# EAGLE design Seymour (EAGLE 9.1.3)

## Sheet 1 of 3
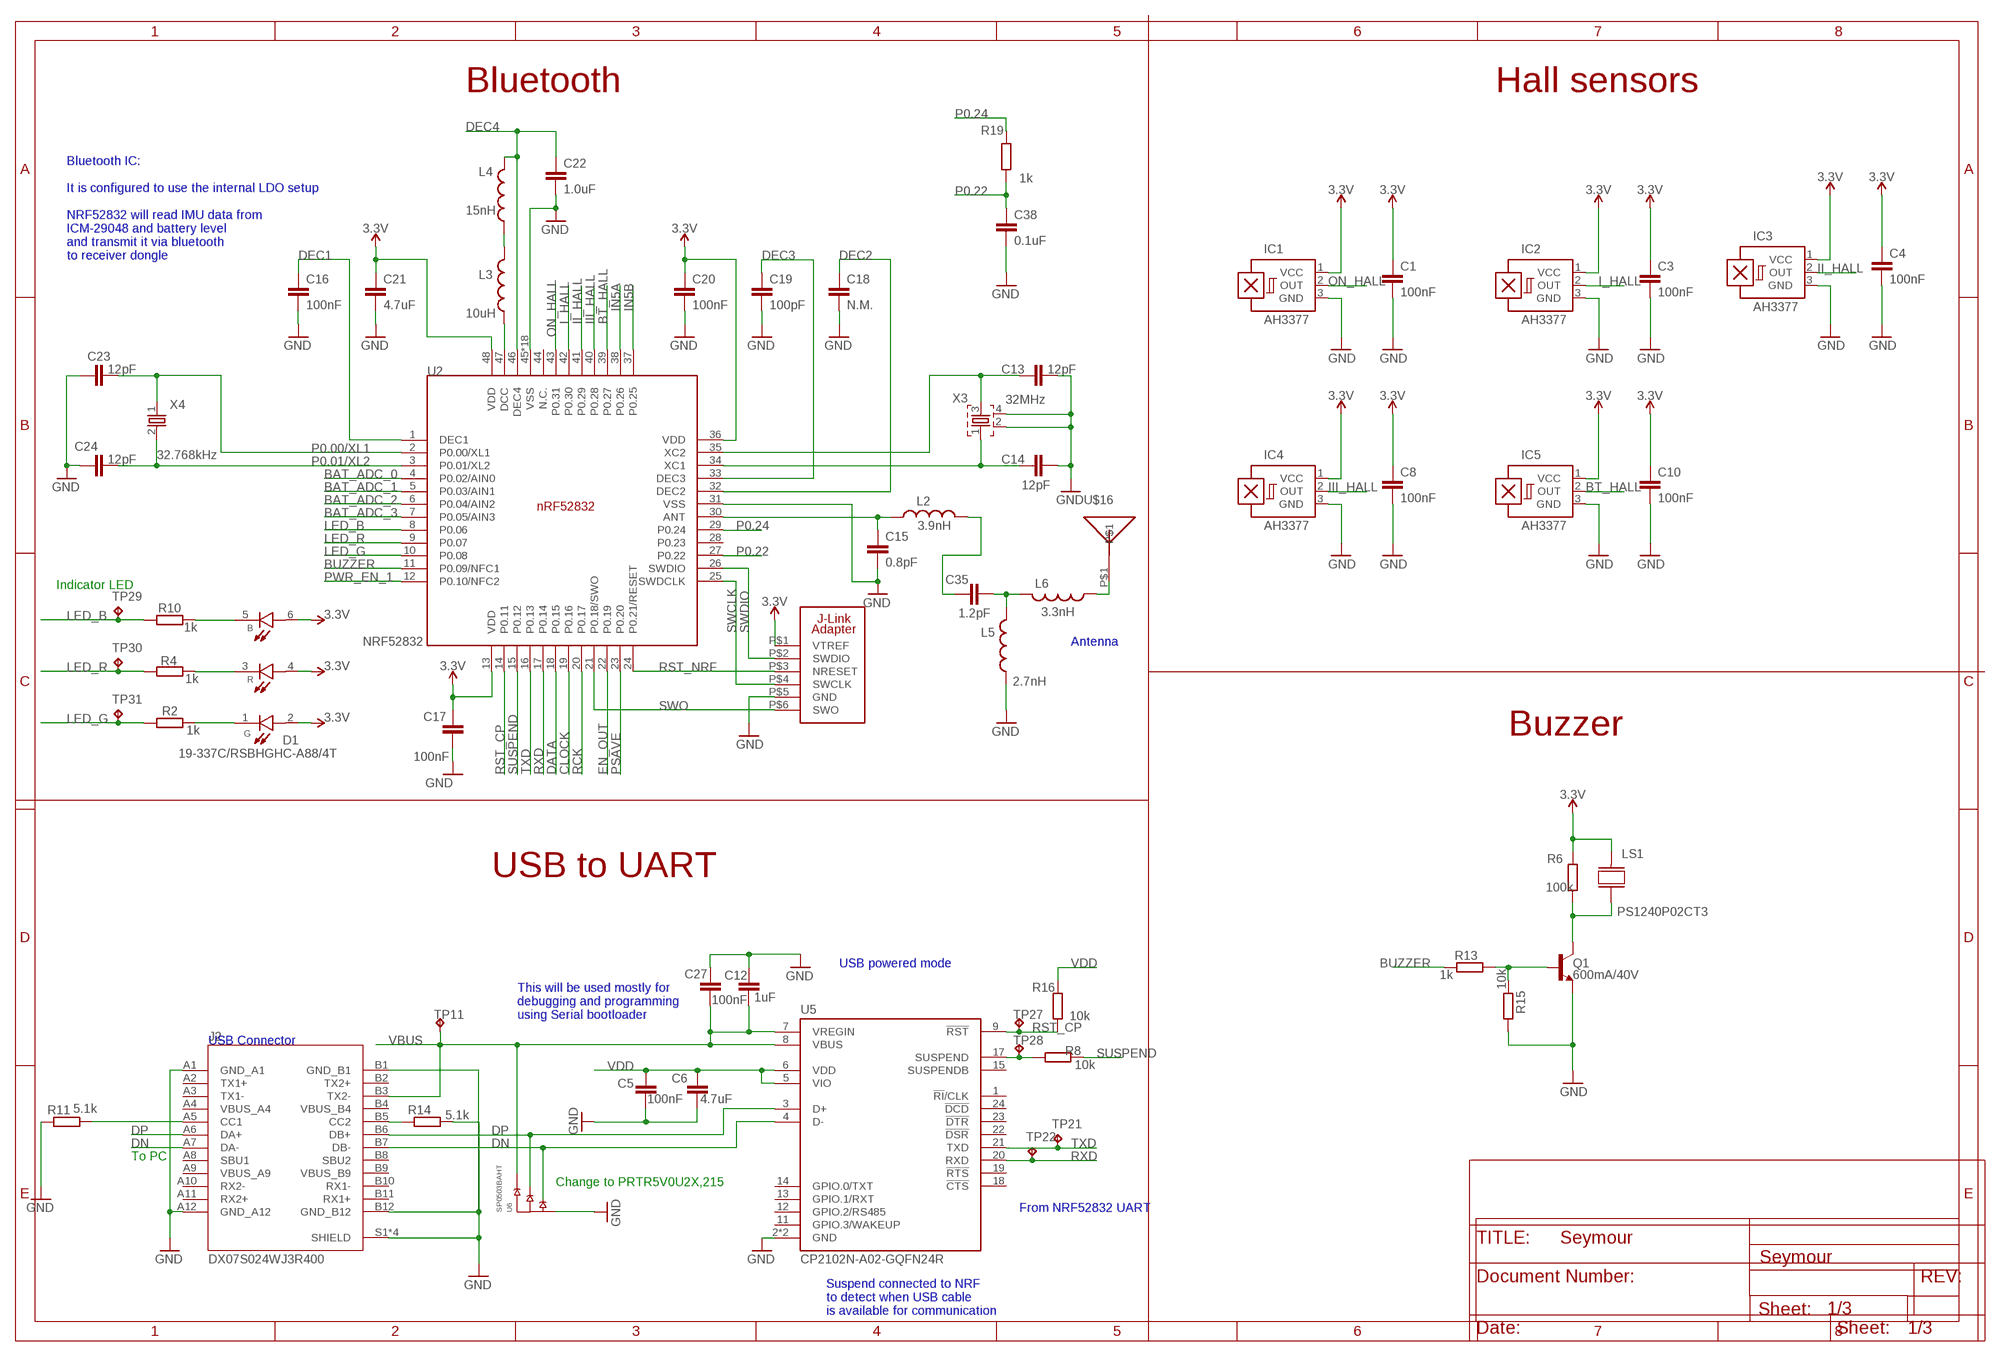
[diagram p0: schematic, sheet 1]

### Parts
C1  100nF  C-EUC0402  [C0402]
C3  100nF  C-EUC0402  [C0402]
C4  100nF  C-EUC0402  [C0402]
C5  100nF  C-EUC0402  [C0402]
C6  4.7uF  C-EUC0603  [C0603]
C8  100nF  C-EUC0402  [C0402]
C10  100nF  C-EUC0402  [C0402]
C12  1uF  C-EUC0603  [C0603]
C13  12pF  C-EUC0402  [C0402]
C14  12pF  C-EUC0402  [C0402]
C15  0.8pF  C-EUC0402  [C0402]
C16  100nF  C-EUC0603  [C0603]
C17  100nF  C-EUC0402  [C0402]
C18  N.M.  C-EUC0603  [C0603]
C19  100pF  C-EUC0402  [C0402]
C20  100nF  C-EUC0402  [C0402]
C21  4.7uF  C-EUC0603  [C0603]
C22  1.0uF  C-EUC0603  [C0603]
C23  12pF  C-EUC0402  [C0402]
C24  12pF  C-EUC0402  [C0402]
C27  100nF  C-EUC0402  [C0402]
C35  1.2pF  CAPACITOR_0402_N  [RESC0402_N]
C38  0.1uF  C-EUC0402  [C0402]
D1  19-337C/RSBHGHC-A88/4T  [LED_19-337C/RSBHGHC-A88/4T]
IC1  AH3377  A1203LH  [SOT23-W]
IC2  AH3377  A1203LH  [SOT23-W]
IC3  AH3377  A1203LH  [SOT23-W]
IC4  AH3377  A1203LH  [SOT23-W]
IC5  AH3377  A1203LH  [SOT23-W]
J2  DX07S024WJ3R400  [JAE_DX07S024WJ3R400]
L2  3.9nH  INDUCTOR_0402_N  [RESC0402_N]
L3  10uH  INDUCTOR_0603_N  [RESC0603_N]
L4  15nH  INDUCTOR_0402_N  [RESC0402_N]
L5  2.7nH  INDUCTOR_0402_N  [RESC0402_N]
L6  3.3nH  INDUCTOR_0402_N  [RESC0402_N]
LS1  PS1240P02CT3  [XDCR_PS1240P02CT3]
Q1  600mA/40V  TRANS_NPN-MMBT2222AL  [SOT23-3]
R2  1k  R-EU_R0402  [R0402]
R4  1k  R-EU_R0402  [R0402]
R6  100k  R-EU_R0402  [R0402]
R8  10k  R-EU_R0402  [R0402]
R10  1k  R-EU_R0402  [R0402]
R11  5.1k  R-EU_R0402  [R0402]
R13  1k  R-EU_R0402  [R0402]
R14  5.1k  R-EU_R0402  [R0402]
R15  10k  R-EU_R0402  [R0402]
R16  10k  R-EU_R0402  [R0402]
R19  1k  R-EU_R0402  [R0402]
TP11  TPTP06R  [TP06R]
TP21  TPTP06R  [TP06R]
TP22  TPTP06R  [TP06R]
TP27  TPTP06R  [TP06R]
TP28  TPTP06R  [TP06R]
TP29  TPTP06R  [TP06R]
TP30  TPTP06R  [TP06R]
TP31  TPTP06R  [TP06R]
U2  NRF52832  [QFN40P600X600X90-48_N]
U5  CP2102N-A02-GQFN24R  [QFN50P400X400X80-25N]
U6  SP0503BAHT  [SOT143]
U$1  J-LINK_6-PIN_ADAPTER-1  [J-LINK_6-PIN_ADAPTER_S]
U$16  ANT_2450AT18B100E  [2450AT18B100E]
X3  32MHz  XTAL_32MHZ  [BT-XTAL_2016_N]
X4  32.768kHz  XTAL_32KHZ  [XTAL_3215_N]

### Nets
3.3V: C1.1 C3.1 C4.1 C8.1 C10.1 C17.1 C20.1 C21.1 D1.2(G_A) D1.4(R_A) D1.6(B_A) IC1.1(VCC) IC2.1(VCC) IC3.1(VCC) IC4.1(VCC) IC5.1(VCC) LS1.2 R6.1 U2.13(VDD) U2.36(VDD) U2.48(VDD) U$1.P$1(VTREF) ; also sheet 2
ANT1: C15.1 L2.1 U2.30(ANT)
BAT_ADC_0: U2.4(P0.02/AIN0) ; also sheet 3
BAT_ADC_1: U2.5(P0.03/AIN1) ; also sheet 3
BAT_ADC_2: U2.6(P0.04/AIN2) ; also sheet 3
BAT_ADC_3: U2.7(P0.05/AIN3) ; also sheet 3
BT_HALL: IC5.2(OUT) U2.39(P0.27)
BUZZER: R13.1 U2.11(P0.09/NFC1)
CLOCK: U2.19(P0.16) ; also sheet 2
DATA: U2.18(P0.15) ; also sheet 2
DEC1: C16.1 U2.1(DEC1)
DEC2: C18.1 U2.32(DEC2)
DEC3: C19.1 U2.33(DEC3)
DEC4: C22.1 L4.2 U2.46(DEC4)
DN: J2.A7(DA-) J2.B7(DB-) U5.4(D-) U6.2(A)
DP: J2.A6(DA+) J2.B6(DB+) U5.3(D+) U6.3(B)
EN_OUT: U2.22(P0.19) ; also sheet 2
GND: C1.2 C3.2 C4.2 C5.1 C6.2 C8.2 C10.2 C12.1 C13.2 C14.2 C15.2 C16.2 C17.2 C18.2 C19.2 C20.2 C21.2 C22.2 C23.1 C24.1 C27.2 C38.2 IC1.3(GND) IC2.3(GND) IC3.3(GND) IC4.3(GND) IC5.3(GND) J2.A1(GND_A1) J2.A12(GND_A12) J2.B1(GND_B1) J2.B12(GND_B12) J2.S1(SHIELD) J2.S2(SHIELD) J2.S3(SHIELD) J2.S4(SHIELD) L5.1 Q1.2(E) R11.1 R14.2 R15.2 U2.31(VSS) U2.45(VSS) U2.PAD(VSS) U2.PAD@VIA01(VSS) U2.PAD@VIA02(VSS) U2.PAD@VIA03(VSS) U2.PAD@VIA04(VSS) U2.PAD@VIA05(VSS) U2.PAD@VIA06(VSS) U2.PAD@VIA07(VSS) U2.PAD@VIA08(VSS) U2.PAD@VIA09(VSS) U2.PAD@VIA10(VSS) U2.PAD@VIA11(VSS) U2.PAD@VIA12(VSS) U2.PAD@VIA13(VSS) U2.PAD@VIA14(VSS) U2.PAD@VIA15(VSS) U2.PAD@VIA16(VSS) U5.2(GND) U5.25(GND) U6.1(GND) U$1.P$5(GND) X3.2 X3.4 ; also sheet 2,3
I_HALL: IC2.2(OUT) U2.42(P0.30)
II_HALL: IC3.2(OUT) U2.41(P0.29)
III_HALL: IC4.2(OUT) U2.40(P0.28)
IN5A: U2.38(P0.26) ; also sheet 2
IN5B: U2.37(P0.25) ; also sheet 2
LED_B: R10.2 TP29.TP U2.8(P0.06)
LED_G: R2.2 TP31.TP U2.10(P0.08)
LED_R: R4.2 TP30.TP U2.9(P0.07) ; also sheet 3
N$1: C13.1 U2.35(XC2) X3.3
N$2: C35.2 L2.2
N$3: R8.1 TP28.TP U5.17(SUSPEND)
N$4: J2.A5(CC1) R11.2
N$5: J2.B5(CC2) R14.1
N$8: D1.3(R_C) R4.1
N$10: D1.5(B_C) R10.1
N$14: Q1.1(B) R13.2 R15.1
N$15: D1.1(G_C) R2.1
N$16: LS1.1 Q1.3(C) R6.2
N$17: L3.1 U2.47(DCC)
N$20: L3.2 L4.1
N$29: C35.1 L5.2 L6.2
N$30: L6.1 U$16.P$1
ON_HALL: IC1.2(OUT) U2.43(P0.31)
P0.00/XL1: C23.2 U2.2(P0.00/XL1) X4.1
P0.01/XL2: C24.2 U2.3(P0.01/XL2) X4.2
P0.22: C38.1 R19.1 U2.27(P0.22)
P0.24: R19.2 U2.29(P0.24)
PSAVE: U2.23(P0.20) ; also sheet 2
PWR_EN_1: U2.12(P0.10/NFC2) ; also sheet 2
RCK: U2.20(P0.17) ; also sheet 2
RST_CP: R16.2 TP27.TP U2.14(P0.11) U5.9(!RST)
RST_NRF: U2.24(P0.21/RESET) U$1.P$3(NRESET)
RXD: TP22.TP U2.17(P0.14) U5.20(RXD)
SUSPEND: R8.2 U2.15(P0.12)
SWCLK: U2.25(SWDCLK) U$1.P$4(SWCLK)
SWDIO: U2.26(SWDIO) U$1.P$2(SWDIO)
SWO: U2.21(P0.18/SWO) U$1.P$6(SWO)
TXD: TP21.TP U2.16(P0.13) U5.21(TXD)
VBUS: C12.2 C27.1 J2.B3(TX2-) TP11.TP U5.7(VREGIN) U5.8(VBUS) U6.4(C) ; also sheet 3
VDD: C5.2 C6.1 R16.1 U5.5(VIO) U5.6(VDD)
X2: C14.1 U2.34(XC1) X3.1
Unconnected: J2.A2(TX1+) J2.A3(TX1-) J2.A4(VBUS_A4) J2.A8(SBU1) J2.A9(VBUS_A9) J2.A10(RX2-) J2.A11(RX2+) J2.B2(TX2+) J2.B4(VBUS_B4) J2.B8(SBU2) J2.B9(VBUS_B9) J2.B10(RX1-) J2.B11(RX1+) U2.28(P0.23) U2.44(N.C.) U5.1(!RI!/CLK) U5.11(GPIO.3/WAKEUP) U5.12(GPIO.2/RS485) U5.13(GPIO.1/RXT) U5.14(GPIO.0/TXT) U5.15(SUSPENDB) U5.18(!CTS) U5.19(!RTS) U5.22(!DSR) U5.23(!DTR) U5.24(!DCD)

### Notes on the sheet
- Bluetooth | Hall sensors
- 1k
- Bluetooth IC:
  
  It is configured to use the internal LDO setup
  
  NRF52832 will read IMU data from 
  ICM-29048 and battery level 
  and transmit it via bluetooth 
  to receiver dongle
- Indicator LED
- Antenna
- Buzzer
- USB to UART
- USB powered mode
- This will be used mostly for 
  debugging and programming 
  using Serial bootloader
- USB Connector
- To PC
- Change to PRTR5V0U2X,215‎
- From NRF52832 UART
- Suspend connected to NRF 
  to detect when USB cable 
  is available for communication

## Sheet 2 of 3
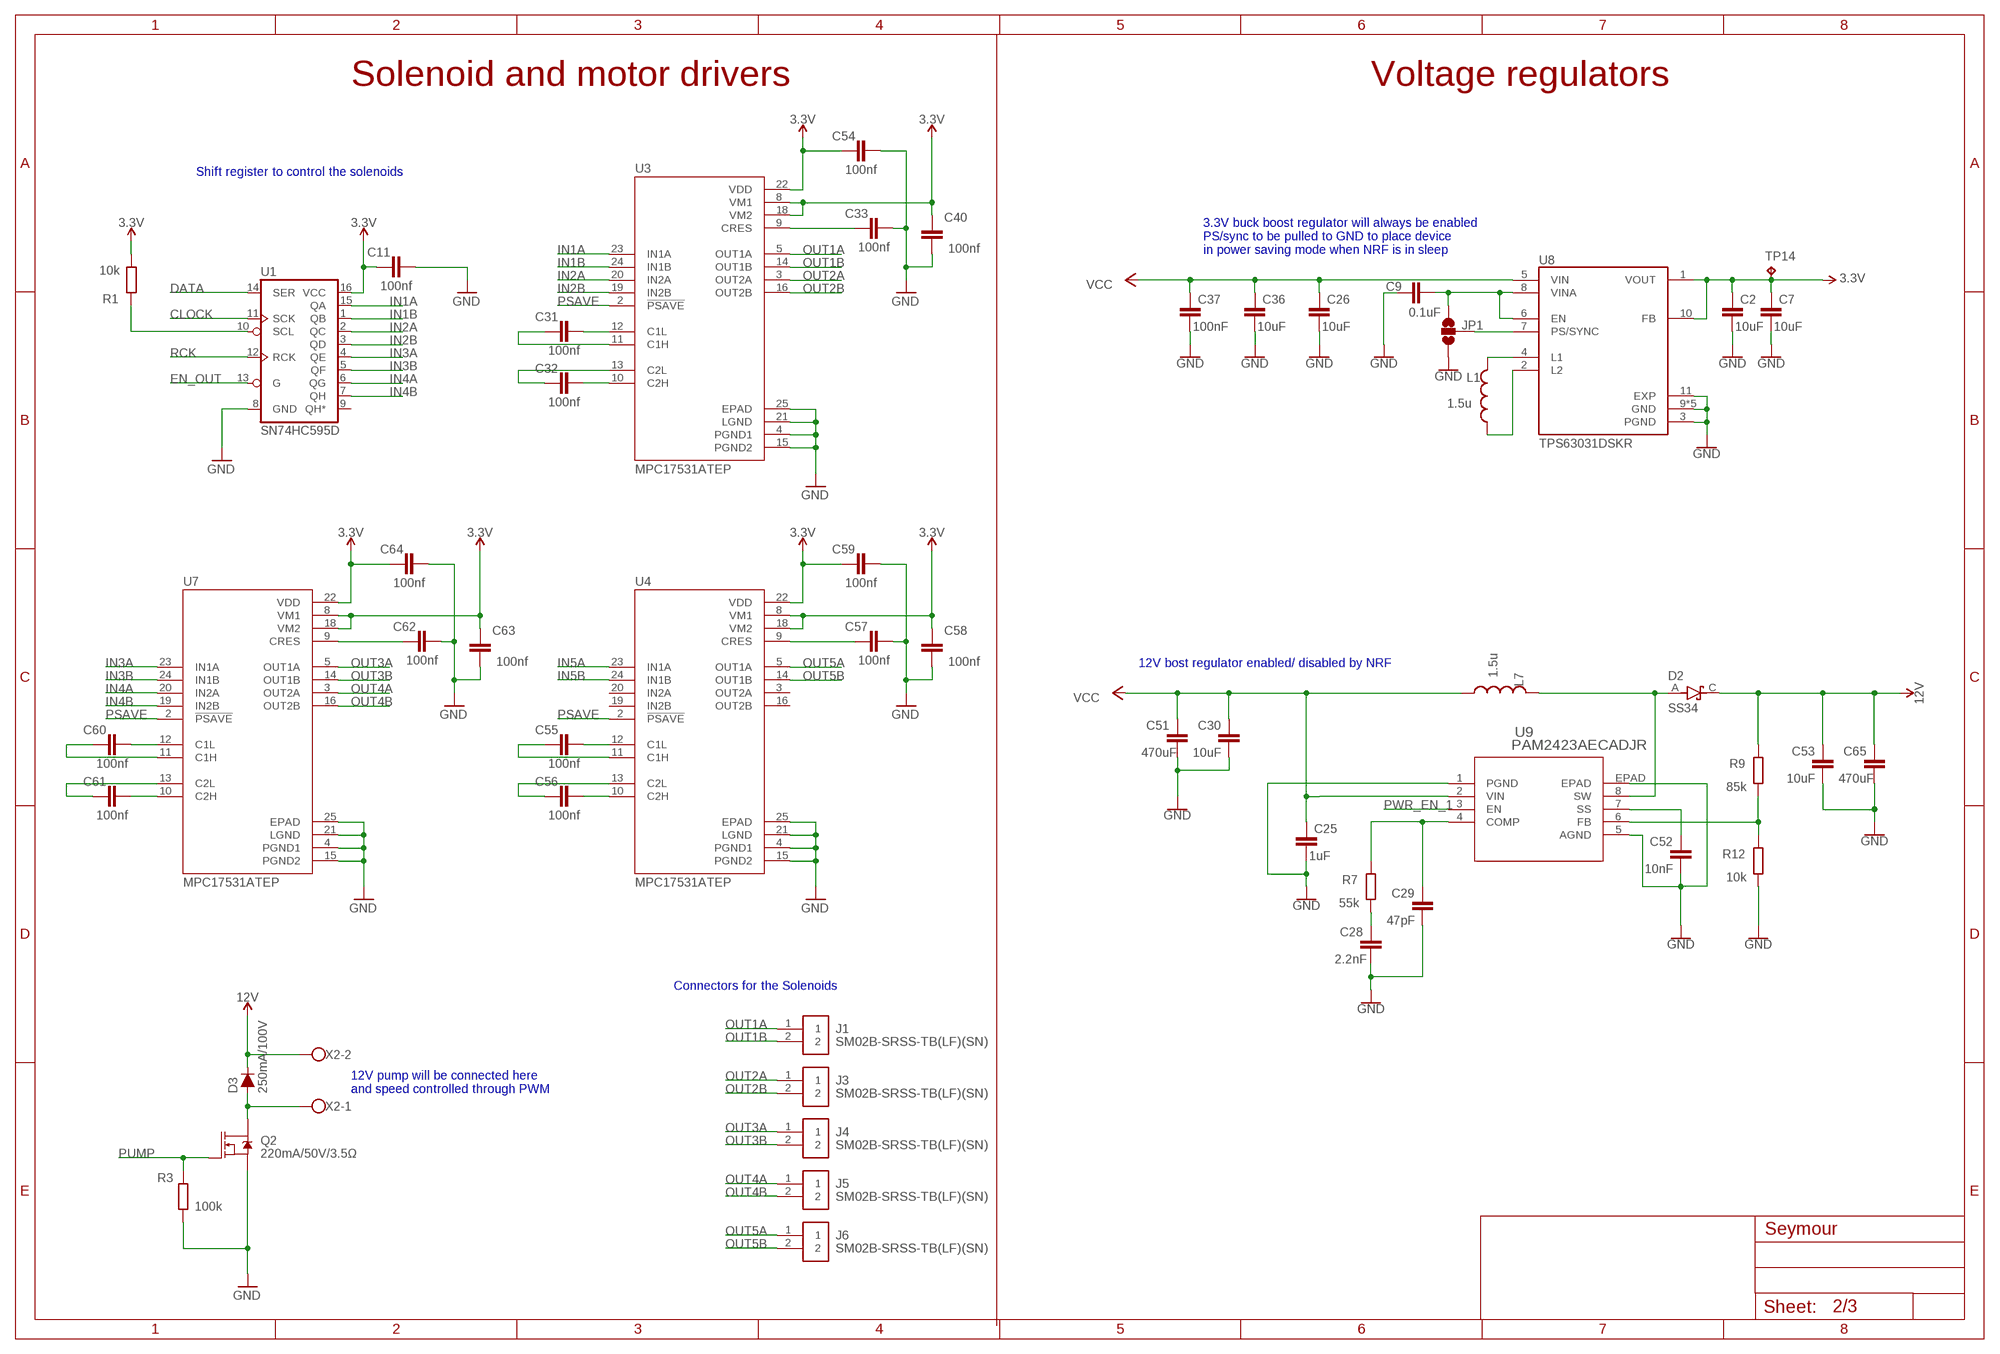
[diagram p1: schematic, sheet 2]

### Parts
C2  10uF  C-EUC0603  [C0603]
C7  10uF  C-EUC0603  [C0603]
C9  0.1uF  C-EUC0603  [C0603]
C11  100nf  CAPACITOR_0402_N  [RESC0402_N]
C25  1uF  C-EUC0603  [C0603]
C26  10uF  C-EUC0603  [C0603]
C28  2.2nF  C-EUC0603  [C0603]
C29  47pF  C-EUC0603  [C0603]
C30  10uF  C-EUC0603  [C0603]
C31  100nf  CAPACITOR_0402_N  [RESC0402_N]
C32  100nf  CAPACITOR_0402_N  [RESC0402_N]
C33  100nf  CAPACITOR_0402_N  [RESC0402_N]
C36  10uF  C-EUC0603  [C0603]
C37  100nF  C-EUC0603  [C0603]
C40  100nf  CAPACITOR_0402_N  [RESC0402_N]
C51  470uF  C-EUC0603  [C0603]
C52  10nF  C-EUC0603  [C0603]
C53  10uF  C-EUC0603  [C0603]
C54  100nf  CAPACITOR_0402_N  [RESC0402_N]
C55  100nf  CAPACITOR_0402_N  [RESC0402_N]
C56  100nf  CAPACITOR_0402_N  [RESC0402_N]
C57  100nf  CAPACITOR_0402_N  [RESC0402_N]
C58  100nf  CAPACITOR_0402_N  [RESC0402_N]
C59  100nf  CAPACITOR_0402_N  [RESC0402_N]
C60  100nf  CAPACITOR_0402_N  [RESC0402_N]
C61  100nf  CAPACITOR_0402_N  [RESC0402_N]
C62  100nf  CAPACITOR_0402_N  [RESC0402_N]
C63  100nf  CAPACITOR_0402_N  [RESC0402_N]
C64  100nf  CAPACITOR_0402_N  [RESC0402_N]
C65  470uF  C-EUC0603  [C0603]
D2  SS34  [DIOM7959X265N]
D3  250mA/100V  DIODE-BAS16J  [SOD-323]
J1  SM02B-SRSS-TB(LF)(SN)  [SM02B-SRSS-TB(LF)(SN)]
J3  SM02B-SRSS-TB(LF)(SN)  [SM02B-SRSS-TB(LF)(SN)]
J4  SM02B-SRSS-TB(LF)(SN)  [SM02B-SRSS-TB(LF)(SN)]
J5  SM02B-SRSS-TB(LF)(SN)  [SM02B-SRSS-TB(LF)(SN)]
J6  SM02B-SRSS-TB(LF)(SN)  [SM02B-SRSS-TB(LF)(SN)]
JP1  SPARKFUN-JUMPERS_JUMPER-SMT_NC  [SPARKFUN-JUMPERS_SMT-JUMPER_TRACE_SILK]
L1  1.5u  XFL4020  [XFL4020]
L7  1.5u  XFL4020  [XFL4020]
Q2  220mA/50V/3.5Ω  MOSFET-NCH-BSS138  [SOT23-3]
R1  10k  R-EU_R0402  [R0402]
R3  100k  R-EU_R0402  [R0402]
R7  55k  R-EU_R0402  [R0402]
R9  85k  R-EU_R0402  [R0402]
R12  10k  R-EU_R0402  [R0402]
TP14  TPTP06R  [TP06R]
U1  SN74HC595D  74HC595D  [SO16]
U3  MPC17531ATEP  [QFN50P400X400X100-25N]
U4  MPC17531ATEP  [QFN50P400X400X100-25N]
U7  MPC17531ATEP  [QFN50P400X400X100-25N]
U8  TPS63031DSKR  [SON50P250X250X80-11N]
U9  PAM2423AECADJR  [SOP-8_PAM2423AECADJR_DIO]
X2  W237-102  [W237-102]

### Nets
3.3V: C2.1 C7.1 C11.2 C40.1 C54.2 C58.1 C59.2 C63.1 C64.2 R1.2 TP14.TP U1.16(VCC) U3.8(VM1) U3.18(VM2) U3.22(VDD) U4.8(VM1) U4.18(VM2) U4.22(VDD) U7.8(VM1) U7.18(VM2) U7.22(VDD) U8.1(VOUT) U8.10(FB) ; also sheet 1
12V: C53.1 C65.1 D2.C(K) D3.C R9.2 X2.2
CLOCK: U1.11(SCK) ; also sheet 1
DATA: U1.14(SER) ; also sheet 1
EN_OUT: U1.13(G) ; also sheet 1
GND: C2.2 C7.2 C9.1 C11.1 C25.2 C26.2 C28.2 C29.2 C30.2 C33.1 C36.2 C37.2 C40.2 C51.2 C52.2 C53.2 C54.1 C57.1 C58.2 C59.1 C62.1 C63.2 C64.1 C65.2 JP1.1 Q2.2(S) R3.2 R12.1 U1.8(GND) U3.4(PGND1) U3.15(PGND2) U3.21(LGND) U3.25(EPAD) U4.4(PGND1) U4.15(PGND2) U4.21(LGND) U4.25(EPAD) U7.4(PGND1) U7.15(PGND2) U7.21(LGND) U7.25(EPAD) U8.3(PGND) U8.9(GND) U8.11(EXP) U8.12(GND) U8.13(GND) U8.14(GND) U8.15(GND) U9.1(PGND) U9.5(AGND) U9.EPAD ; also sheet 1,3
IN1A: U1.15(QA) U3.23(IN1A)
IN1B: U1.1(QB) U3.24(IN1B)
IN2A: U1.2(QC) U3.20(IN2A)
IN2B: U1.3(QD) U3.19(IN2B)
IN3A: U1.4(QE) U7.23(IN1A)
IN3B: U1.5(QF) U7.24(IN1B)
IN4A: U1.6(QG) U7.20(IN2A)
IN4B: U1.7(QH) U7.19(IN2B)
IN5A: U4.23(IN1A) ; also sheet 1
IN5B: U4.24(IN1B) ; also sheet 1
N$6: C9.2 JP1.3 U8.6(EN) U8.8(VINA)
N$7: L1.P$2 U8.4(L1)
N$9: R1.1 U1.10(SCL)
N$11: L1.P$1 U8.2(L2)
N$12: D2.A L7.P$2 U9.8(SW)
N$13: JP1.2 U8.7(PS/SYNC)
N$18: C29.1 R7.2 U9.4(COMP)
N$19: C28.1 R7.1
N$23: C52.1 U9.7(SS)
N$39: R9.1 R12.2 U9.6(FB)
N$43: C32.1 U3.10(C2H)
N$44: C32.2 U3.13(C2L)
N$45: C31.2 U3.11(C1H)
N$46: C31.1 U3.12(C1L)
N$47: C33.2 U3.9(CRES)
N$48: D3.A Q2.3(D) X2.1
N$51: C56.1 U4.10(C2H)
N$52: C56.2 U4.13(C2L)
N$53: C55.2 U4.11(C1H)
N$54: C55.1 U4.12(C1L)
N$55: C57.2 U4.9(CRES)
N$58: C61.1 U7.10(C2H)
N$59: C61.2 U7.13(C2L)
N$60: C60.2 U7.11(C1H)
N$61: C60.1 U7.12(C1L)
N$62: C62.2 U7.9(CRES)
OUT1A: J1.1 U3.5(OUT1A)
OUT1B: J1.2 U3.14(OUT1B)
OUT2A: J3.1 U3.3(OUT2A)
OUT2B: J3.2 U3.16(OUT2B)
OUT3A: J4.1 U7.5(OUT1A)
OUT3B: J4.2 U7.14(OUT1B)
OUT4A: J5.1 U7.3(OUT2A)
OUT4B: J5.2 U7.16(OUT2B)
OUT5A: J6.1 U4.5(OUT1A)
OUT5B: J6.2 U4.14(OUT1B)
PSAVE: U3.2(!PSAVE) U4.2(!PSAVE) U7.2(!PSAVE) ; also sheet 1
PUMP: Q2.1(G) R3.1
PWR_EN_1: U9.3(EN) ; also sheet 1
RCK: U1.12(RCK) ; also sheet 1
VCC: C25.1 C26.1 C30.1 C36.1 C37.1 C51.1 L7.P$1 U8.5(VIN) U9.2(VIN) ; also sheet 3
Unconnected: U1.9(QH*) U4.3(OUT2A) U4.16(OUT2B) U4.19(IN2B) U4.20(IN2A)

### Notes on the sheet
- Solenoid and motor drivers | Voltage regulators
- Shift register to control the solenoids
- 3.3V buck boost regulator will always be enabled
  PS/sync to be pulled to GND to place device 
  in power saving mode when NRF is in sleep
- 12V bost regulator enabled/ disabled by NRF
- Connectors for the Solenoids
- 12V pump will be connected here 
  and speed controlled through PWM

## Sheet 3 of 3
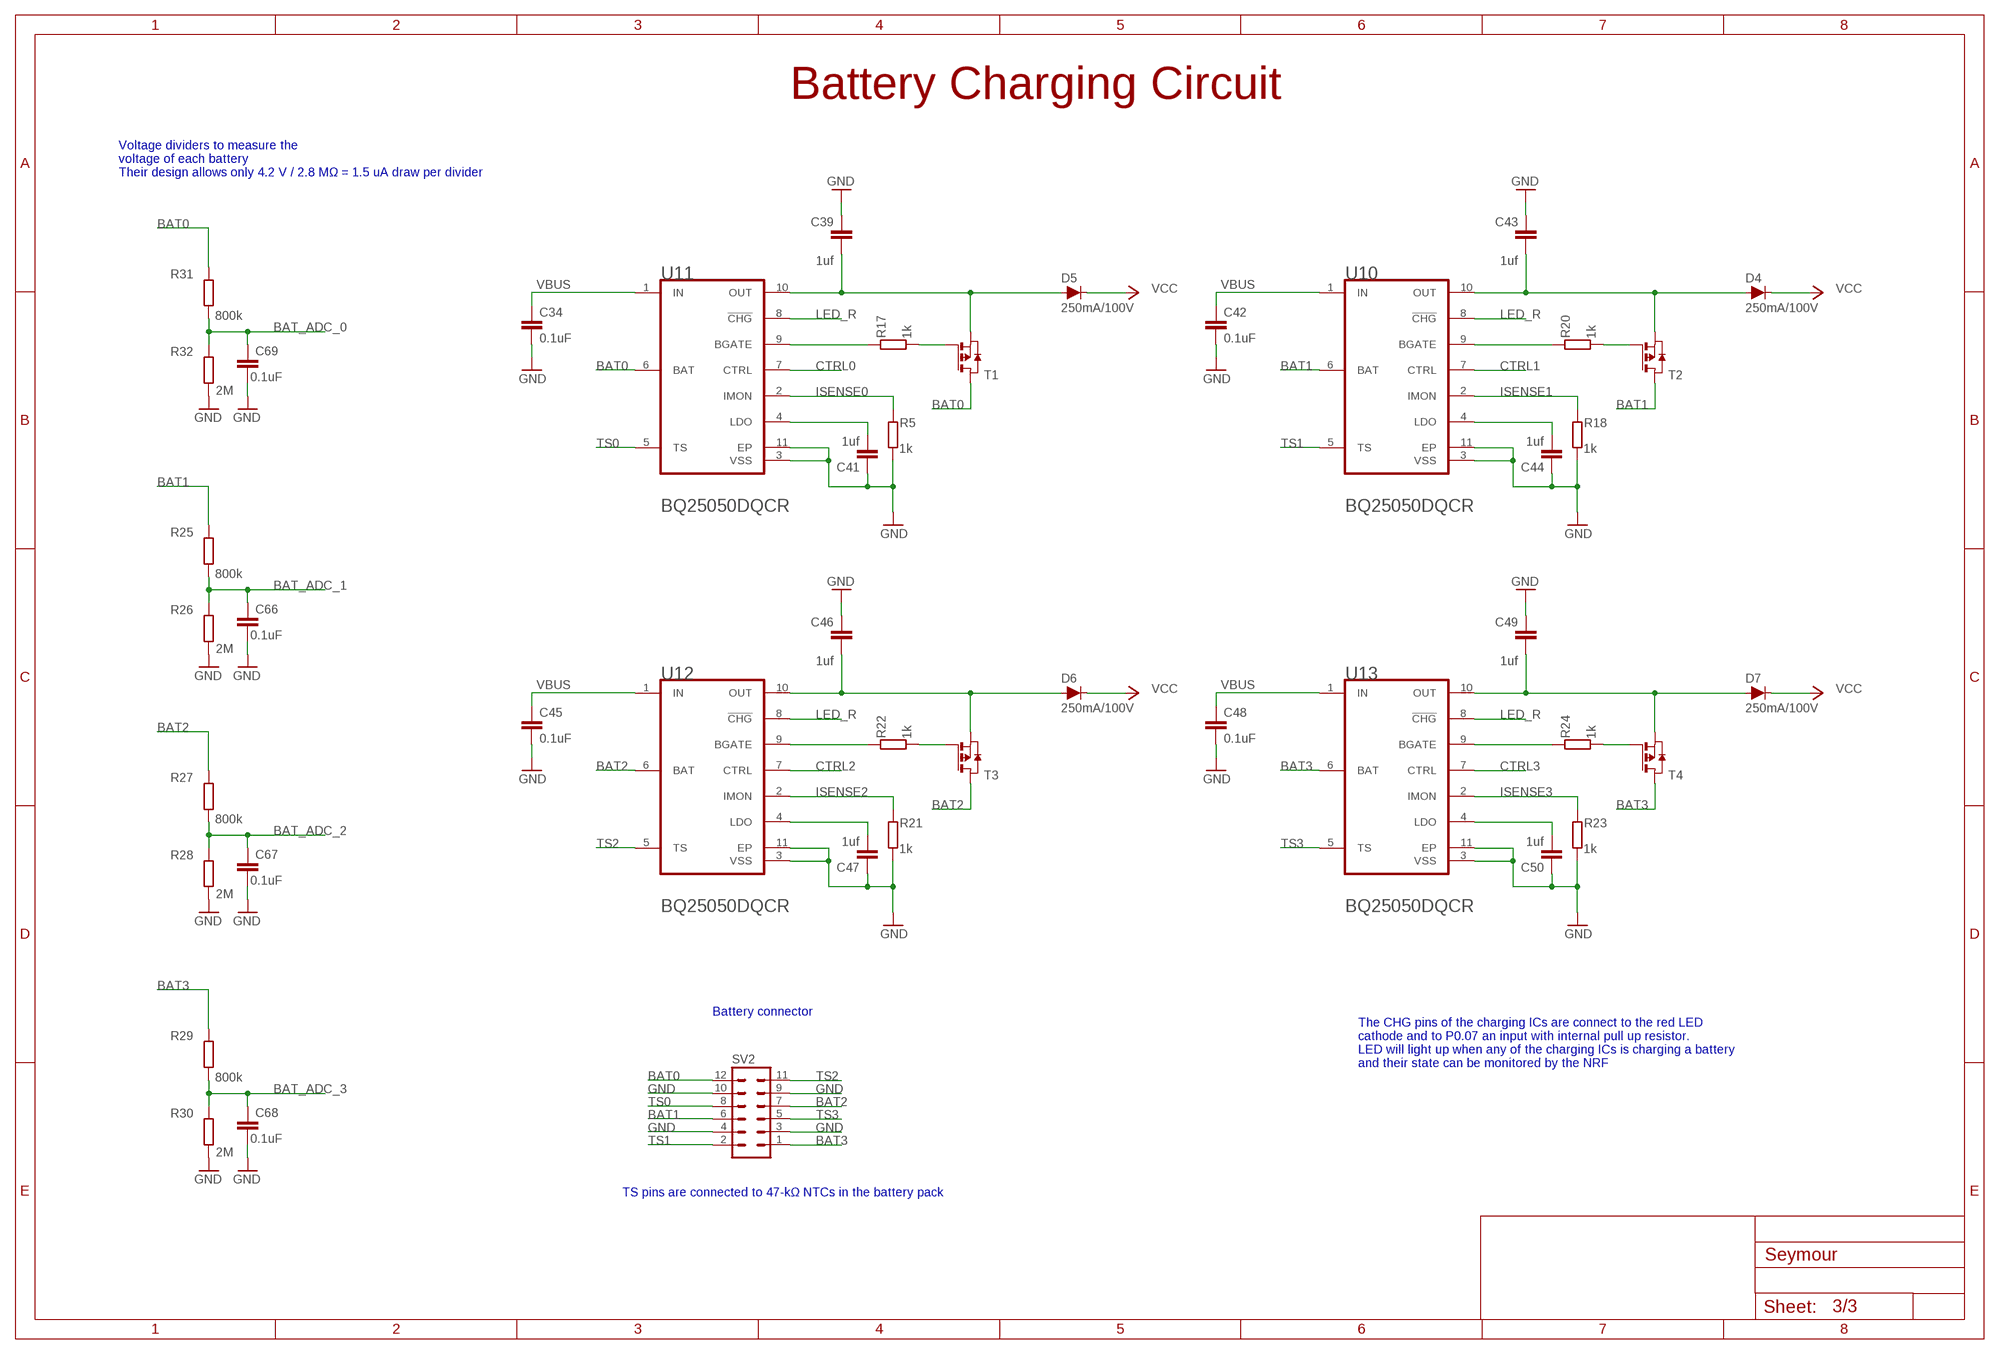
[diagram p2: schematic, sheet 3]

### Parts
C34  0.1uF  C-EUC0402  [C0402]
C39  1uf  C-EUC0402  [C0402]
C41  1uf  C-EUC0402  [C0402]
C42  0.1uF  C-EUC0402  [C0402]
C43  1uf  C-EUC0402  [C0402]
C44  1uf  C-EUC0402  [C0402]
C45  0.1uF  C-EUC0402  [C0402]
C46  1uf  C-EUC0402  [C0402]
C47  1uf  C-EUC0402  [C0402]
C48  0.1uF  C-EUC0402  [C0402]
C49  1uf  C-EUC0402  [C0402]
C50  1uf  C-EUC0402  [C0402]
C66  0.1uF  C-EUC0402  [C0402]
C67  0.1uF  C-EUC0402  [C0402]
C68  0.1uF  C-EUC0402  [C0402]
C69  0.1uF  C-EUC0402  [C0402]
D4  250mA/100V  DIODE-BAS16J  [SOD-323]
D5  250mA/100V  DIODE-BAS16J  [SOD-323]
D6  250mA/100V  DIODE-BAS16J  [SOD-323]
D7  250mA/100V  DIODE-BAS16J  [SOD-323]
R5  1k  R-EU_R0402  [R0402]
R17  1k  R-EU_R0402  [R0402]
R18  1k  R-EU_R0402  [R0402]
R20  1k  R-EU_R0402  [R0402]
R21  1k  R-EU_R0402  [R0402]
R22  1k  R-EU_R0402  [R0402]
R23  1k  R-EU_R0402  [R0402]
R24  1k  R-EU_R0402  [R0402]
R25  800k  R-EU_R0402  [R0402]
R26  2M  R-EU_R0402  [R0402]
R27  800k  R-EU_R0402  [R0402]
R28  2M  R-EU_R0402  [R0402]
R29  800k  R-EU_R0402  [R0402]
R30  2M  R-EU_R0402  [R0402]
R31  800k  R-EU_R0402  [R0402]
R32  2M  R-EU_R0402  [R0402]
SV2  MA06-2  [MA06-2]
T1  PMOSSOT23  [SOT-23]
T2  PMOSSOT23  [SOT-23]
T3  PMOSSOT23  [SOT-23]
T4  PMOSSOT23  [SOT-23]
U10  TEXAS_INSTRUMENTS_BQ25050DQCRTEXAS_INSTRUMENTS_BQ25050DQCR_0_0  [TEXAS_INSTRUMENTS_BQ25050DQCR_0]
U11  TEXAS_INSTRUMENTS_BQ25050DQCRTEXAS_INSTRUMENTS_BQ25050DQCR_0_0  [TEXAS_INSTRUMENTS_BQ25050DQCR_0]
U12  TEXAS_INSTRUMENTS_BQ25050DQCRTEXAS_INSTRUMENTS_BQ25050DQCR_0_0  [TEXAS_INSTRUMENTS_BQ25050DQCR_0]
U13  TEXAS_INSTRUMENTS_BQ25050DQCRTEXAS_INSTRUMENTS_BQ25050DQCR_0_0  [TEXAS_INSTRUMENTS_BQ25050DQCR_0]

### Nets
BAT0: R31.2 SV2.12 T1.1(D) U11.6(BAT)
BAT1: R25.2 SV2.6 T2.1(D) U10.6(BAT)
BAT2: R27.2 SV2.7 T3.1(D) U12.6(BAT)
BAT3: R29.2 SV2.1 T4.1(D) U13.6(BAT)
BAT_ADC_0: C69.1 R31.1 R32.2 ; also sheet 1
BAT_ADC_1: C66.1 R25.1 R26.2 ; also sheet 1
BAT_ADC_2: C67.1 R27.1 R28.2 ; also sheet 1
BAT_ADC_3: C68.1 R29.1 R30.2 ; also sheet 1
CTRL0: U11.7(CTRL)
CTRL1: U10.7(CTRL)
CTRL2: U12.7(CTRL)
CTRL3: U13.7(CTRL)
GND: C34.2 C39.1 C41.1 C42.2 C43.1 C44.1 C45.2 C46.1 C47.1 C48.2 C49.1 C50.1 C66.2 C67.2 C68.2 C69.2 R5.1 R18.1 R21.1 R23.1 R26.1 R28.1 R30.1 R32.1 SV2.3 SV2.4 SV2.9 SV2.10 U10.3(VSS) U10.11(EP) U11.3(VSS) U11.11(EP) U12.3(VSS) U12.11(EP) U13.3(VSS) U13.11(EP) ; also sheet 1,2
ISENSE0: R5.2 U11.2(IMON)
ISENSE1: R18.2 U10.2(IMON)
ISENSE2: R21.2 U12.2(IMON)
ISENSE3: R23.2 U13.2(IMON)
LED_R: U10.8(!CHG!) U11.8(!CHG!) U12.8(!CHG!) U13.8(!CHG!) ; also sheet 1
N$21: R17.1 T1.3(G)
N$24: R17.2 U11.9(BGATE)
N$26: C39.2 D5.A T1.2(S) U11.10(OUT)
N$27: C44.2 U10.4(LDO)
N$28: C41.2 U11.4(LDO)
N$31: C43.2 D4.A T2.2(S) U10.10(OUT)
N$33: R20.2 U10.9(BGATE)
N$34: R20.1 T2.3(G)
N$36: C47.2 U12.4(LDO)
N$37: C46.2 D6.A T3.2(S) U12.10(OUT)
N$40: R22.2 U12.9(BGATE)
N$41: R22.1 T3.3(G)
N$50: C50.2 U13.4(LDO)
N$56: C49.2 D7.A T4.2(S) U13.10(OUT)
N$63: R24.2 U13.9(BGATE)
N$64: R24.1 T4.3(G)
TS0: SV2.8 U11.5(TS)
TS1: SV2.2 U10.5(TS)
TS2: SV2.11 U12.5(TS)
TS3: SV2.5 U13.5(TS)
VBUS: C34.1 C42.1 C45.1 C48.1 U10.1(IN) U11.1(IN) U12.1(IN) U13.1(IN) ; also sheet 1
VCC: D4.C D5.C D6.C D7.C ; also sheet 2

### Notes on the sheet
- Battery Charging Circuit
- Voltage dividers to measure the
  voltage of each battery
  Their design allows only 4.2 V / 2.8 MΩ = 1.5 uA draw per divider
- Battery connector
- The CHG pins of the charging ICs are connect to the red LED
  cathode and to P0.07 an input with internal pull up resistor.
  LED will light up when any of the charging ICs is charging a battery
  and their state can be monitored by the NRF
- TS pins are connected to 47-kΩ NTCs in the battery pack

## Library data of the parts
C1 C3 C4 C8 C10 C17 C20 C34 C39 C41-C50 C66-C69 = rcl:C-EU: CAPACITOR, European symbol; SPICEPREFIX: C
C2 C5-C7 C9 C12-C16 C18 C19 C21-C30 C36-C38 C51-C53 C65 = resistor:C-EU: CAPACITOR, European symbol
C11 C31-C33 C35 C40 C54-C64 = Nordic_nRF:CAPACITOR: Generic chip capacitor
D1 = led:19-337C/RSBHGHC-A88/4T: Red, Green, Blue (RGB) 625nm Red, 530nm Green, 470nm Blue LED Indication - Discrete 2.05V Red, 2.9V Green, 2.9V Blue 0606 (1616 Metric) Check prices; AVAILABILITY: Warning; DESCRIPTION: Red, Green, Blue (RGB) 625nm Red, 530nm Green, 470nm Blue LED Indication - Discrete 2.05V Red, 2.9V Green, 2.9V Blue 0606 (1616 Metric); MF: Everlight Electronics Co Ltd; MP: 19-337C/RSBHGHC-A88/4T; PACKAGE: 0606 Everlight Electronics Co Ltd; PRICE: None; PURCHASE-URL: https://pricing.snapeda.com/search/part/19-337C/RSBHGHC-A88/4T/?ref=eda
D2 = SS34:SS34: Diode Schottky 40V 3A 2-Pin SMC T/R Check prices; AVAILABILITY: In Stock; DESCRIPTION: Diode Schottky 40V 3A Surface Mount SMC (DO-214AB); MF: ON Semiconductor; MP: SS34; PACKAGE: SMC-2 ON Semiconductor; PRICE: None; PURCHASE-URL: https://pricing.snapeda.com/search/part/SS34/?ref=eda
D3-D7 = SparkFun-DiscreteSemi:DIODE: Diode; PROD_ID: DIO-09646
IC1-IC5 = allegro:A12*?: Hall-effect bipolar switch Source: http://www.allegromicro.com/en/Products/Part_Numbers/1202/1202.pdf; MF: ALLEGRO MICROSYSTEMS, INC.; MPN: A1203LLHLT-T; OC_FARNELL: 1791384; OC_NEWARK: 31K6608
J1 J3-J6 = SM02B-SRSS-TB_LF__SN_:SM02B-SRSS-TB(LF)(SN): JST (JAPAN SOLDERLESS TERMINALS) - SM02B-SRSS-TB (LF)(SN) - HEADER, R/A, 2WAY; AVAILABILITY: Unavailable; DESCRIPTION: Connector Header Surface Mount, Right Angle 2 position 0.039 _1.00mm_; MF: JST Sales; MP: SM02B-SRSS-TB_LF__SN_; PACKAGE: None; PRICE: None
J2 = DX07S024WJ3R400:DX07S024WJ3R400: Conn Rcpt Usb3.1 Typec Smd Vert; DESCRIPTION: USB-C (USB TYPE-C) USB 3.2 Gen 2 (USB 3.1 Gen 2, Superspeed + (USB 3.1)) Receptacle Connector 24 Position Surface Mount, Through Hole; DIGI-KEY_PART_NUMBER: 670-2950-1-ND; MF: JAE Electronics; MP: DX07S024WJ3R400; PACKAGE: None; PURCHASE-URL: https://pricing.snapeda.com/search/part/DX07S024WJ3R400/?ref=eda
JP1 = DECAMove:SPARKFUN-JUMPERS_JUMPER-SMT: Normally closed trace jumper (1 of 2 connections) This jumper has a trace between two pads so it's normally closed (NC). The other connection is normally open (NO). Use a razor knife to open the connection. For best results follow the IPC guidelines for cutting traces: Cutout at least 0.063 mm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
L1 L7 = inductor-coilcraft:XFL4020: Coilcraft shielded 4x4mm high temperature inductor
L2-L6 = Nordic_nRF:INDUCTOR: Generic chip inductor
LS1 = PS1240P02CT3:PS1240P02CT3: Buzzers Transducer, Externally Driven Piezo 3V 4kHz 60dB @ 3V, 10cm Through Hole PC Pins; DESCRIPTION: Buzzers Transducer, Externally Driven Piezo 3V 4kHz 60dB @ 3V, 10cm Through Hole PC Pins; DIGI-KEY_PART_NUMBER: 445-5229-1-ND; MF: TDK; MP: PS1240P02CT3; PACKAGE: SIP-5 TDK; PURCHASE-URL: https://pricing.snapeda.com/search/part/PS1240P02CT3/?ref=eda
Q1 = SparkFun-DiscreteSemi:TRANS_NPN: NPN transistor Current controlled devices typically used to amplify current or used as a switch. BC547 - COM-08928 (TO-92 45V 100mA) (1.Collector 2.Base 3.Emitter) 2N3904 - COM-00521 (TO-92 40V 200mA) (1.Emitter 2.Base 3.Collector) P2N2222A - COM-12852 (TO-92 40V 600mA) (1.Collector 2.Base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; PROD_ID: TRANS-08049
Q2 = SparkFun-DiscreteSemi:MOSFET-NCH: N-channel MOSFETs Voltage controlled devices that allow control of high current outputs. SparkFun Products: SparkFun OpenScale SparkFun Digital Sandbox SparkFun Monster Moto Shield SparkFun MOSFET Power Controller; PROD_ID: TRANS-00830
R1-R4 R6-R10 R12 R13 R15 R16 R25-R32 = resistor:R-EU_: RESISTOR, European symbol
R5 R11 R14 R17-R24 = rcl:R-EU_: RESISTOR, European symbol; SPICEPREFIX: R
SV2 = con-lstb:MA06-2: PIN HEADER; OC_FARNELL: unknown; OC_NEWARK: unknown
T1-T4 = zetex:PMOSSOT23: MOS FET; OC_FARNELL: unknown; OC_NEWARK: unknown
TP11 TP14 TP21 TP22 TP27-TP31 = testpad:TP: Test pad
U1 = SparkFun-IC-Logic:74*595: 8-Bit Shift Register (Serial to Parallel) Datasheet SparkFun Products SparkFun Shift Register Breakout - 74HC595 (BOB-10680); PROD_ID: IC-07875
U2 = Nordic_nRF:NRF52832: nRF52832 Features Single chip, highly flexible, 2.4 GHz multi-protocol SoC 32-bit ARM Cortex-M4F Processor 1.7v to 3.6v operation 512kB flash + 64kB RAM Supports concurrent Bluetooth Smart/ANT protocol operation On-chip NFC tag for Out-of-Band (OOB) pairing Up to +4dBm output power -96dBm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
U3 U4 U7 = MPC17531ATEP:MPC17531ATEP: H-Bridge, Dual, Low Voltage, Stepper & DC Brushed Motor Driver, 2-8.6V, 1.4A, 200kHz, QFN 24, Tray Check prices; AVAILABILITY: In Stock; DESCRIPTION: Dual H-Bridge Motor Driver 3V 24-Pin QFN EP Tray; MF: NXP Semiconductors; MP: MPC17531ATEP; PACKAGE: None; PRICE: None; PURCHASE-URL: https://pricing.snapeda.com/search/part/MPC17531ATEP/?ref=eda
U5 = silabs:CP2102N-A02-GQFN24R: Check prices; AVAILABILITY: Warning; DESCRIPTION: USB Bridge, USB to UART USB 2.0 UART Interface 24-QFN (4x4); MF: Silicon Labs; MP: CP2102N-A02-GQFN24R; PACKAGE: WFQFN-24 Silicon Labs; PRICE: None; PURCHASE-URL: https://pricing.snapeda.com/search/part/CP2102N-A02-GQFN24R/?ref=eda
U6 = diode:SP0503BAHT; AVAILABILITY: Unavailable; DESCRIPTION: 8.5V Clamp Ipp Tvs Diode Surface Mount SOT-143-4; MF: Littelfuse Inc.; MP: SP0503BAHT; PACKAGE: SOT-143 Littelfuse; PRICE: None
U8 = TPS63031DSKR:TPS63031DSKR: High Efficient Single Inductor Buck-Boost Converter with 1-A Switches Check prices; AVAILABILITY: Good; DESCRIPTION: High Efficient Single Inductor Buck-Boost Converter with 1-A Switches 10-SON -40 to 85; MF: Texas Instruments; MP: TPS63031DSKR; PACKAGE: WSON-10 Texas Instruments; PRICE: None; PURCHASE-URL: https://pricing.snapeda.com/search/part/TPS63031DSKR/?ref=eda
U9 = PAM2423AECADJR:PAM2423AECADJR; COPYRIGHT: Copyright (C) 2021 Ultra Librarian. All rights reserved.; DIGI-KEY_PART_NUMBER_1: PAM2423AECADJRDITR-ND; DIGI-KEY_PART_NUMBER_2: PAM2423AECADJRDICT-ND; DIGI-KEY_PART_NUMBER_3: PAM2423AECADJRDIDKR-ND; MANUFACTURER_PART_NUMBER: PAM2423AECADJR; MFR_NAME: Diodes Inc
U10-U13 = Texas Instruments - BQ25050DQCR:TEXAS_INSTRUMENTS_BQ25050DQCR: TI-BQ25050DQC10-2400X840TP; DATASHEET: http://www.ti.com/general/docs/lit/getliterature.tsp?genericPartNumber=BQ25050&fileType=pdf; DATASHEET_VERSION: SLUSA33; IMPORTED: yes; IMPORTED_FROM: vault; IMPORT_TS: 1521149580; LEAD_ACID: N; LI__ION: N; LI__POLYMER: N; MF: Texas Instruments; MOUNTING_TECHNOLOGY: Surface Mount; MPN: BQ25050DQCR; NI_CD: N; NI_MH: N; OVER_VOLTAGE_PROTECTION: N; PACKAGE: DQC0010A; PACKAGE_DESCRIPTION: 10-Pin Plastic Small Outline No-Lead, 2 x 3 x 0.8 mm Body, 0.5 mm Pitch, Exposed Pad; PACKAGE_VERSION: revA, Jul-2008; PREFIX: U; ROHS: Yes; SUB_FAMILY: Battery Charge Management; VAULT_GUID: 3EB91702-DF68-4836-8F8E-4B956DA718DA; VAULT_REVISION: C57A6326-882D-4660-8B69-1983E239C76B
U$1 = debug-connectors:J-LINK_6-PIN_ADAPTER: J-Link 6-pin Adapter See https://www.segger.com/jlink-6-pin-adapter.html
U$16 = Johanson_antennas:ANT_2450AT18B100E
X2 = con-wago-500:W237-102: WAGO SCREW CLAMP; MPN: 237-102; OC_FARNELL: unknown; OC_NEWARK: 70K9898
X3 = Nordic_nRF:XTAL_32MHZ
X4 = Nordic_nRF:XTAL_32KHZ

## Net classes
2 lowpower: width 0.254 mm, drill 0.381 mm

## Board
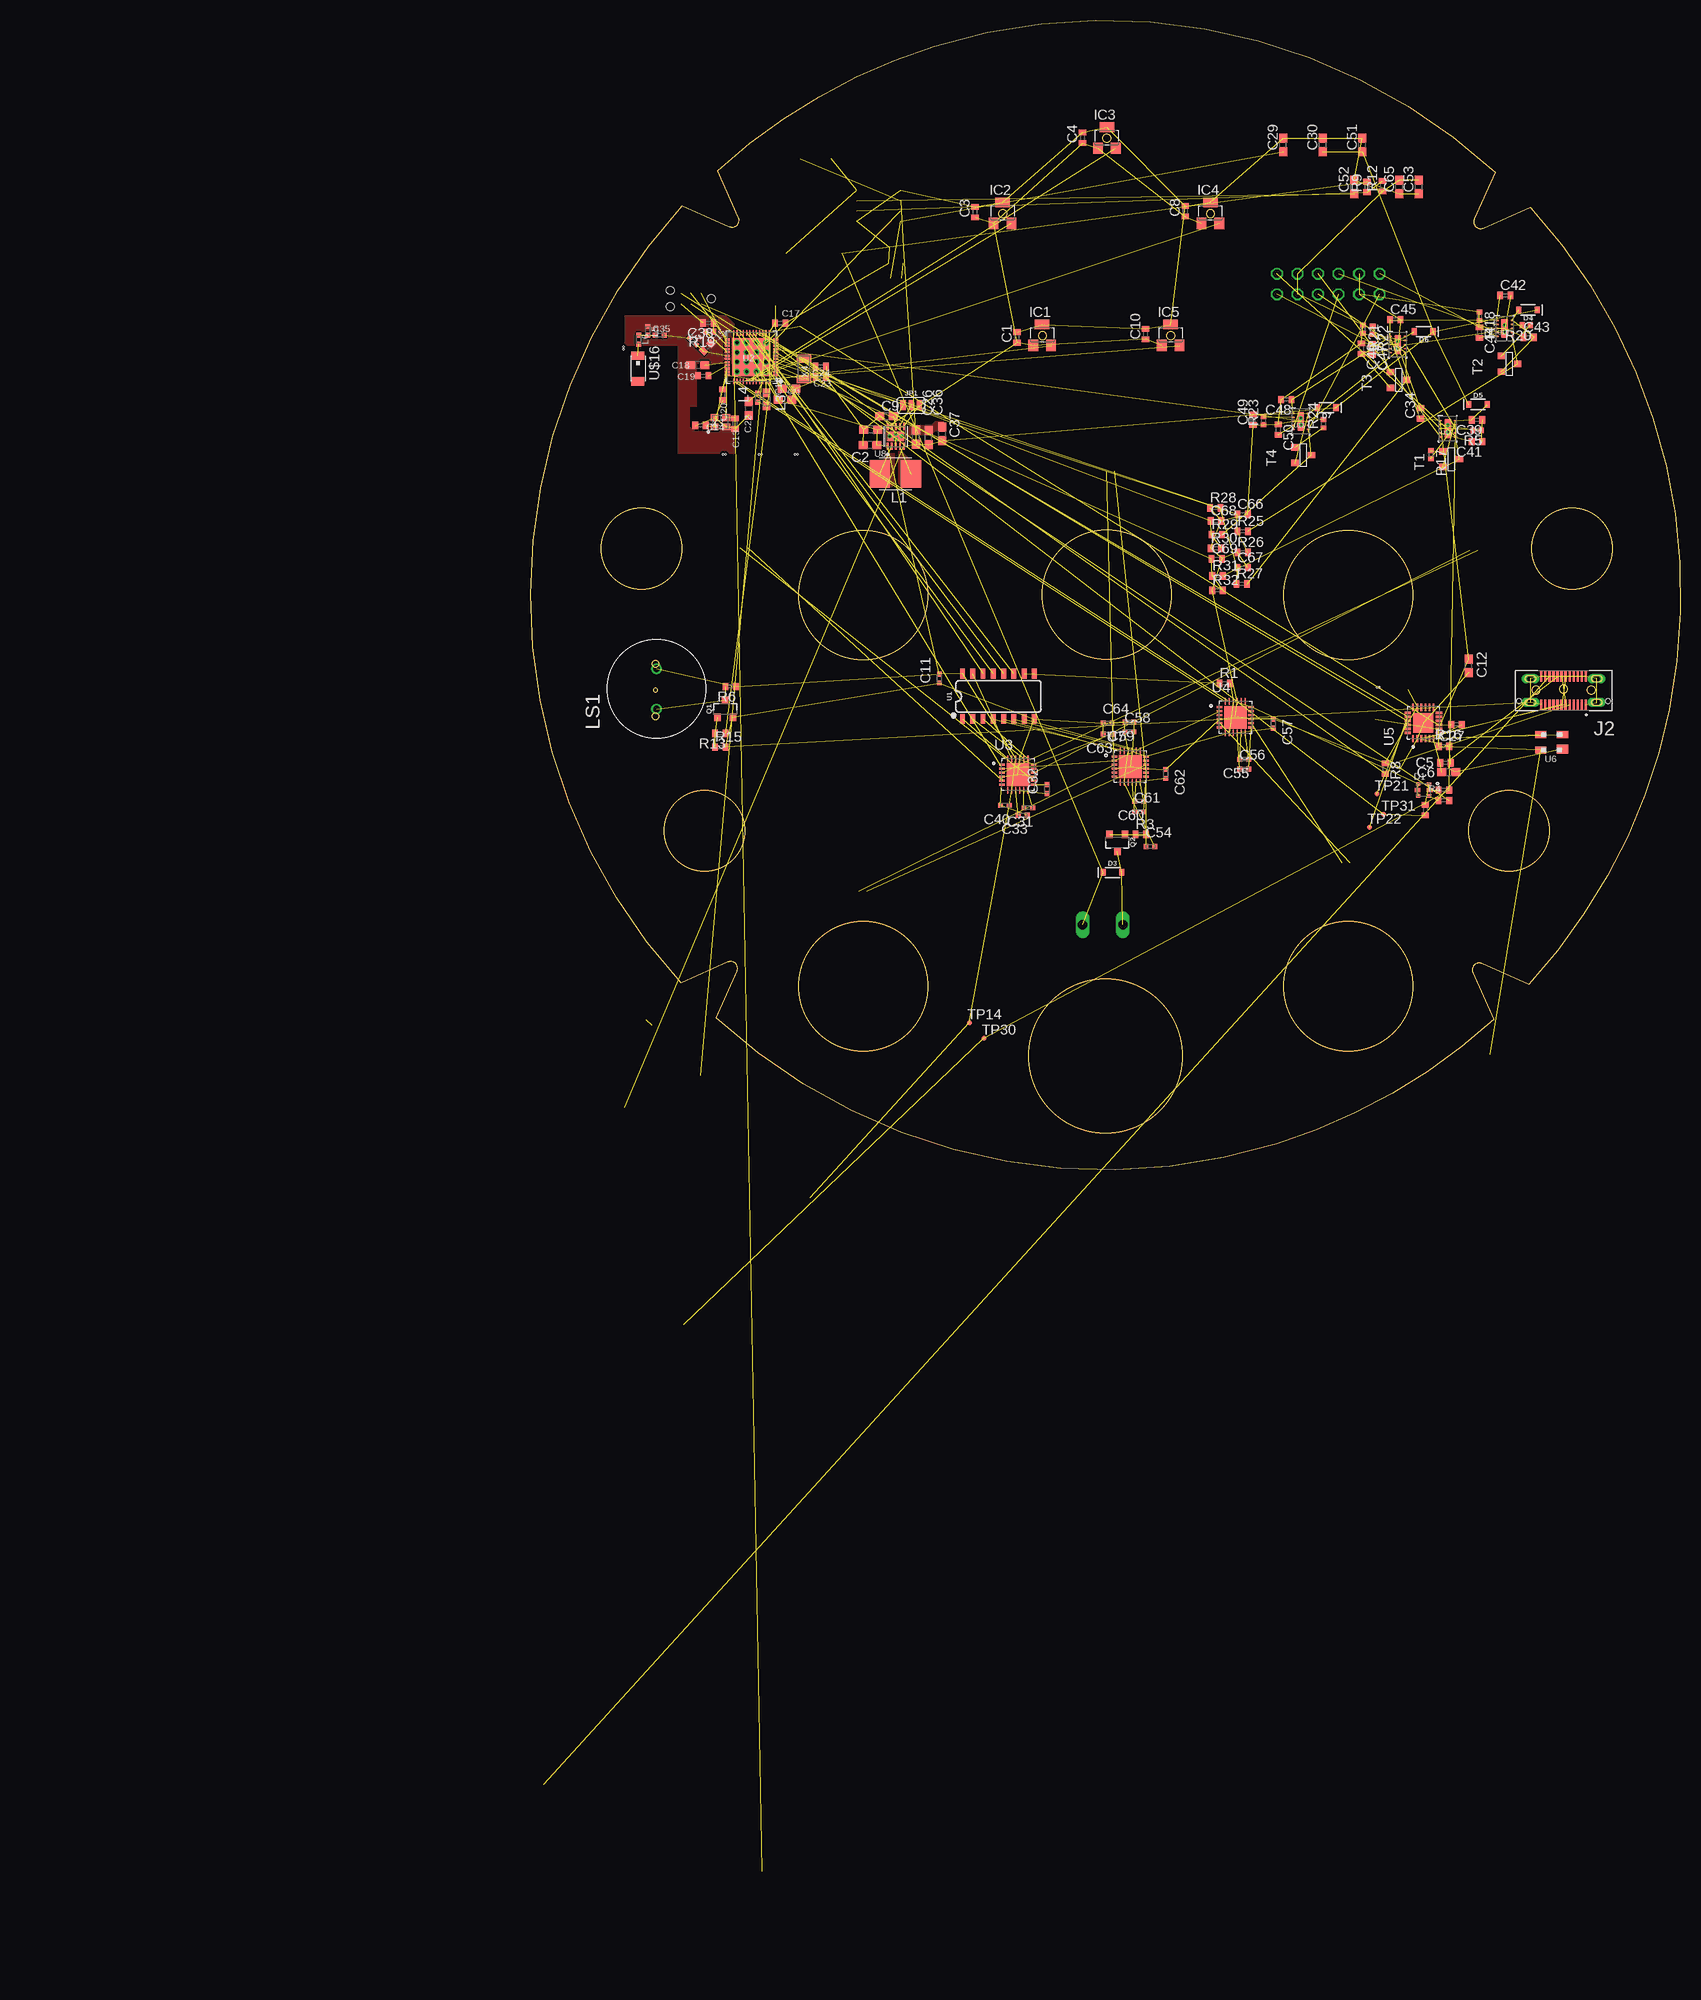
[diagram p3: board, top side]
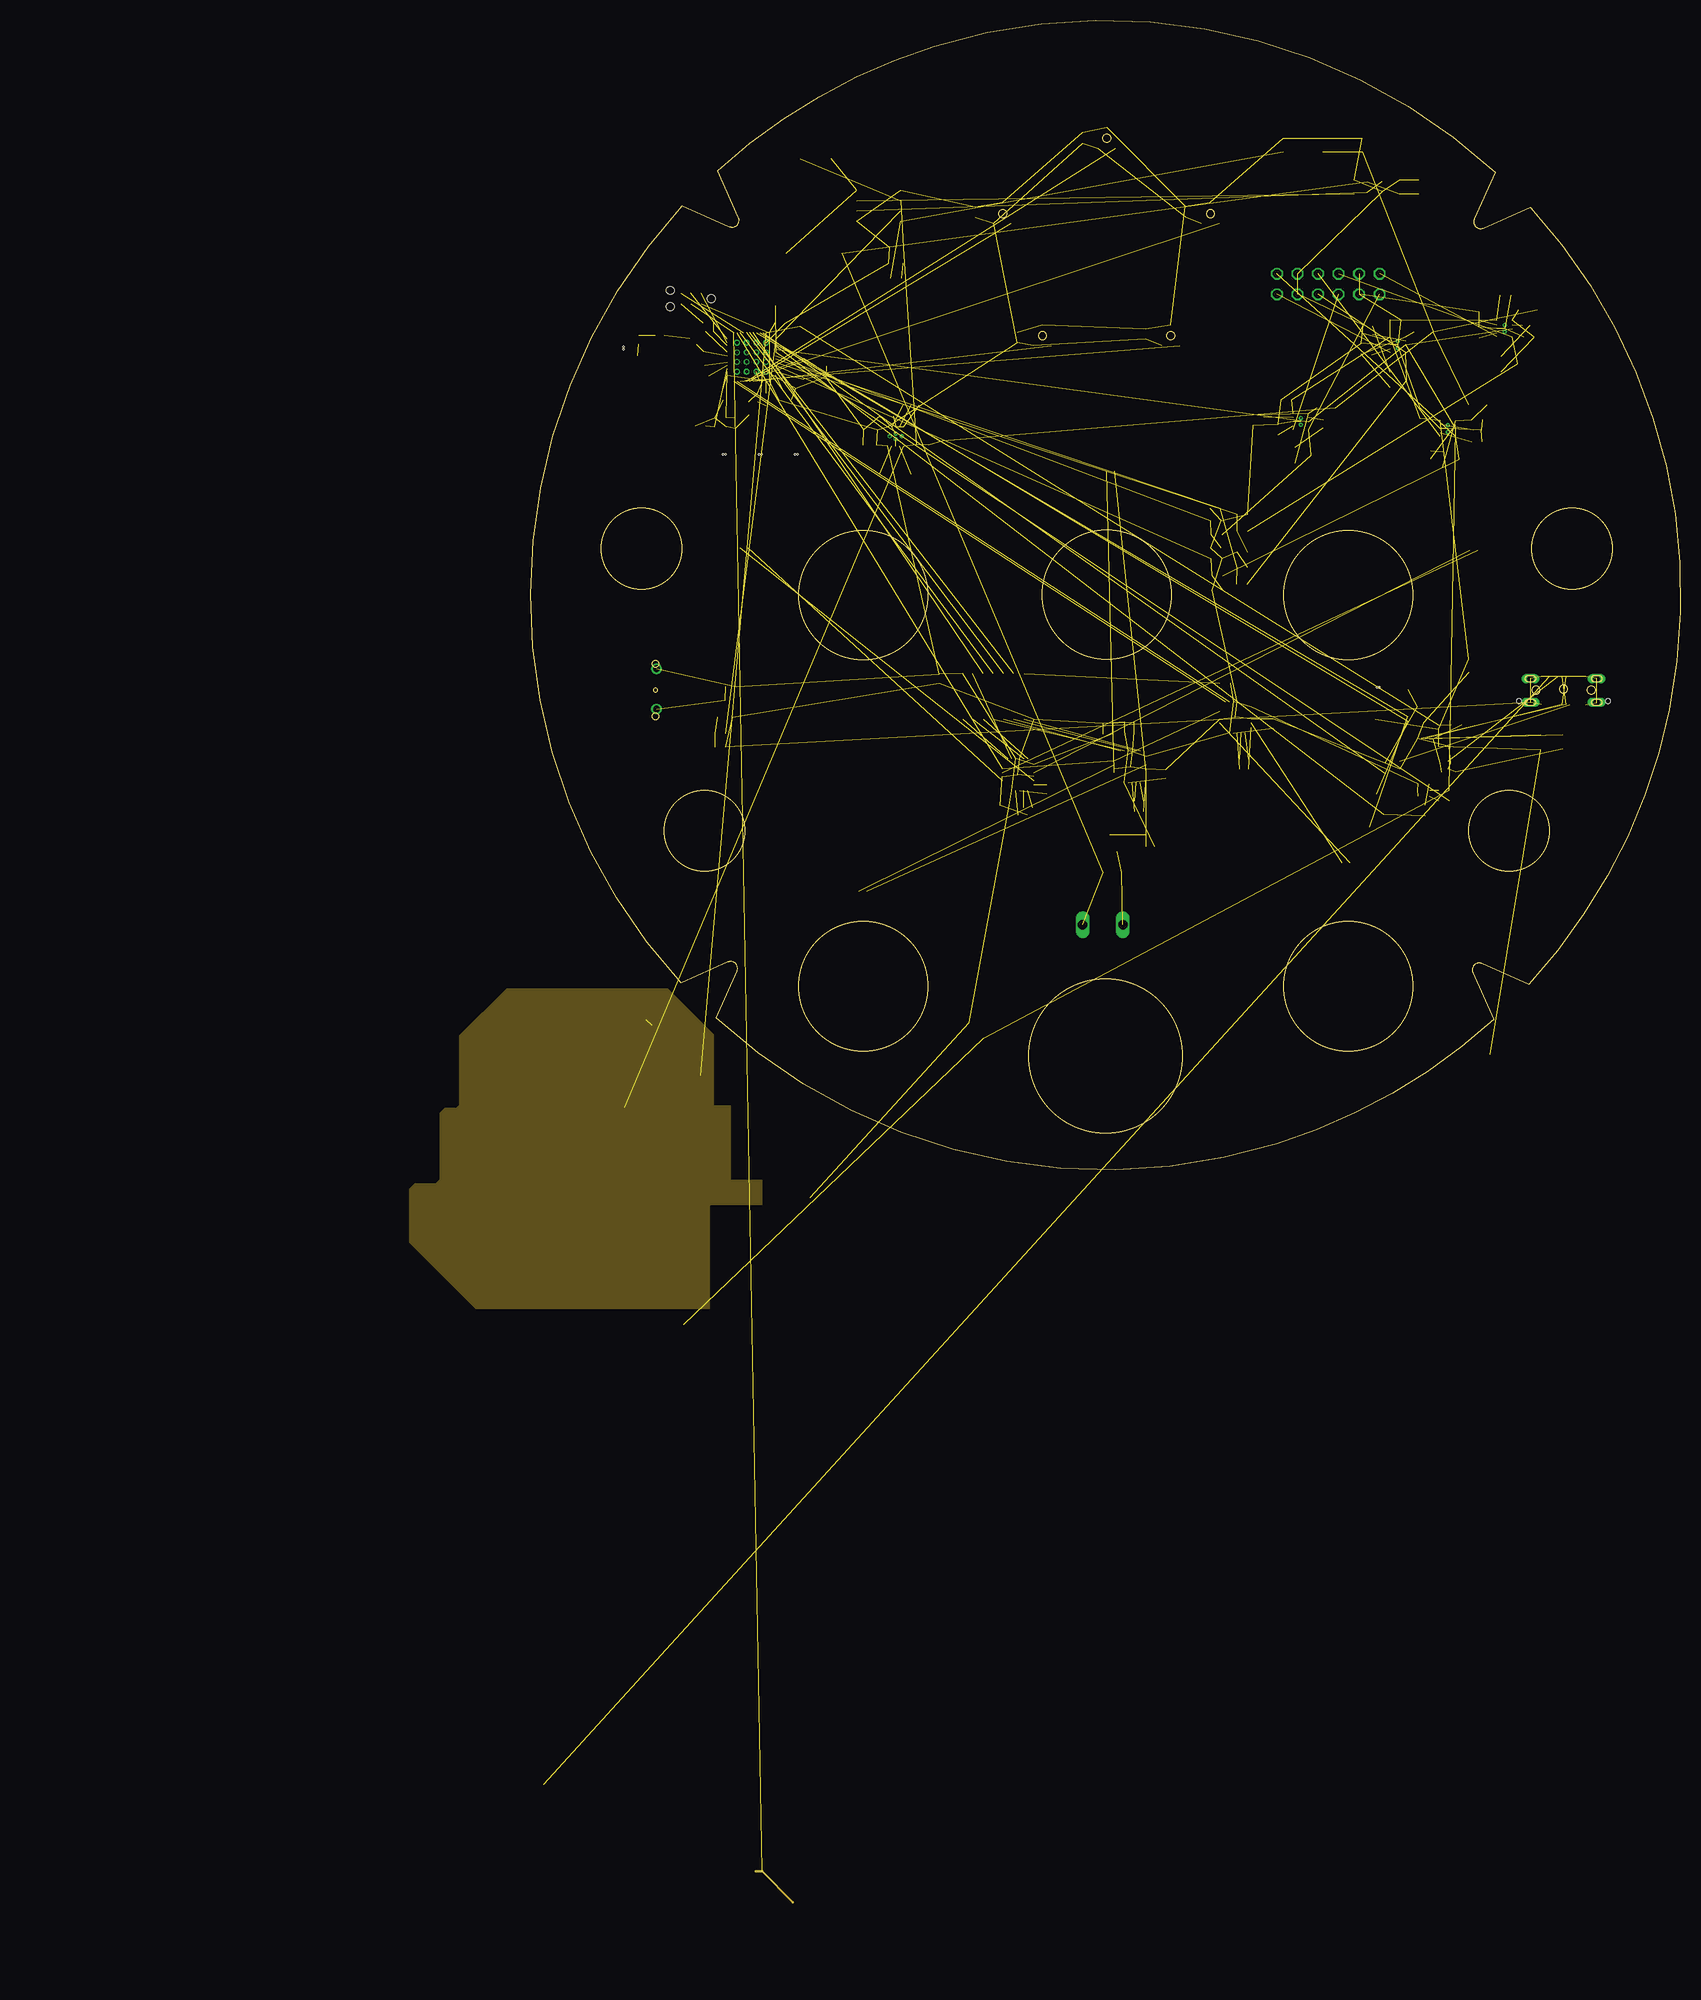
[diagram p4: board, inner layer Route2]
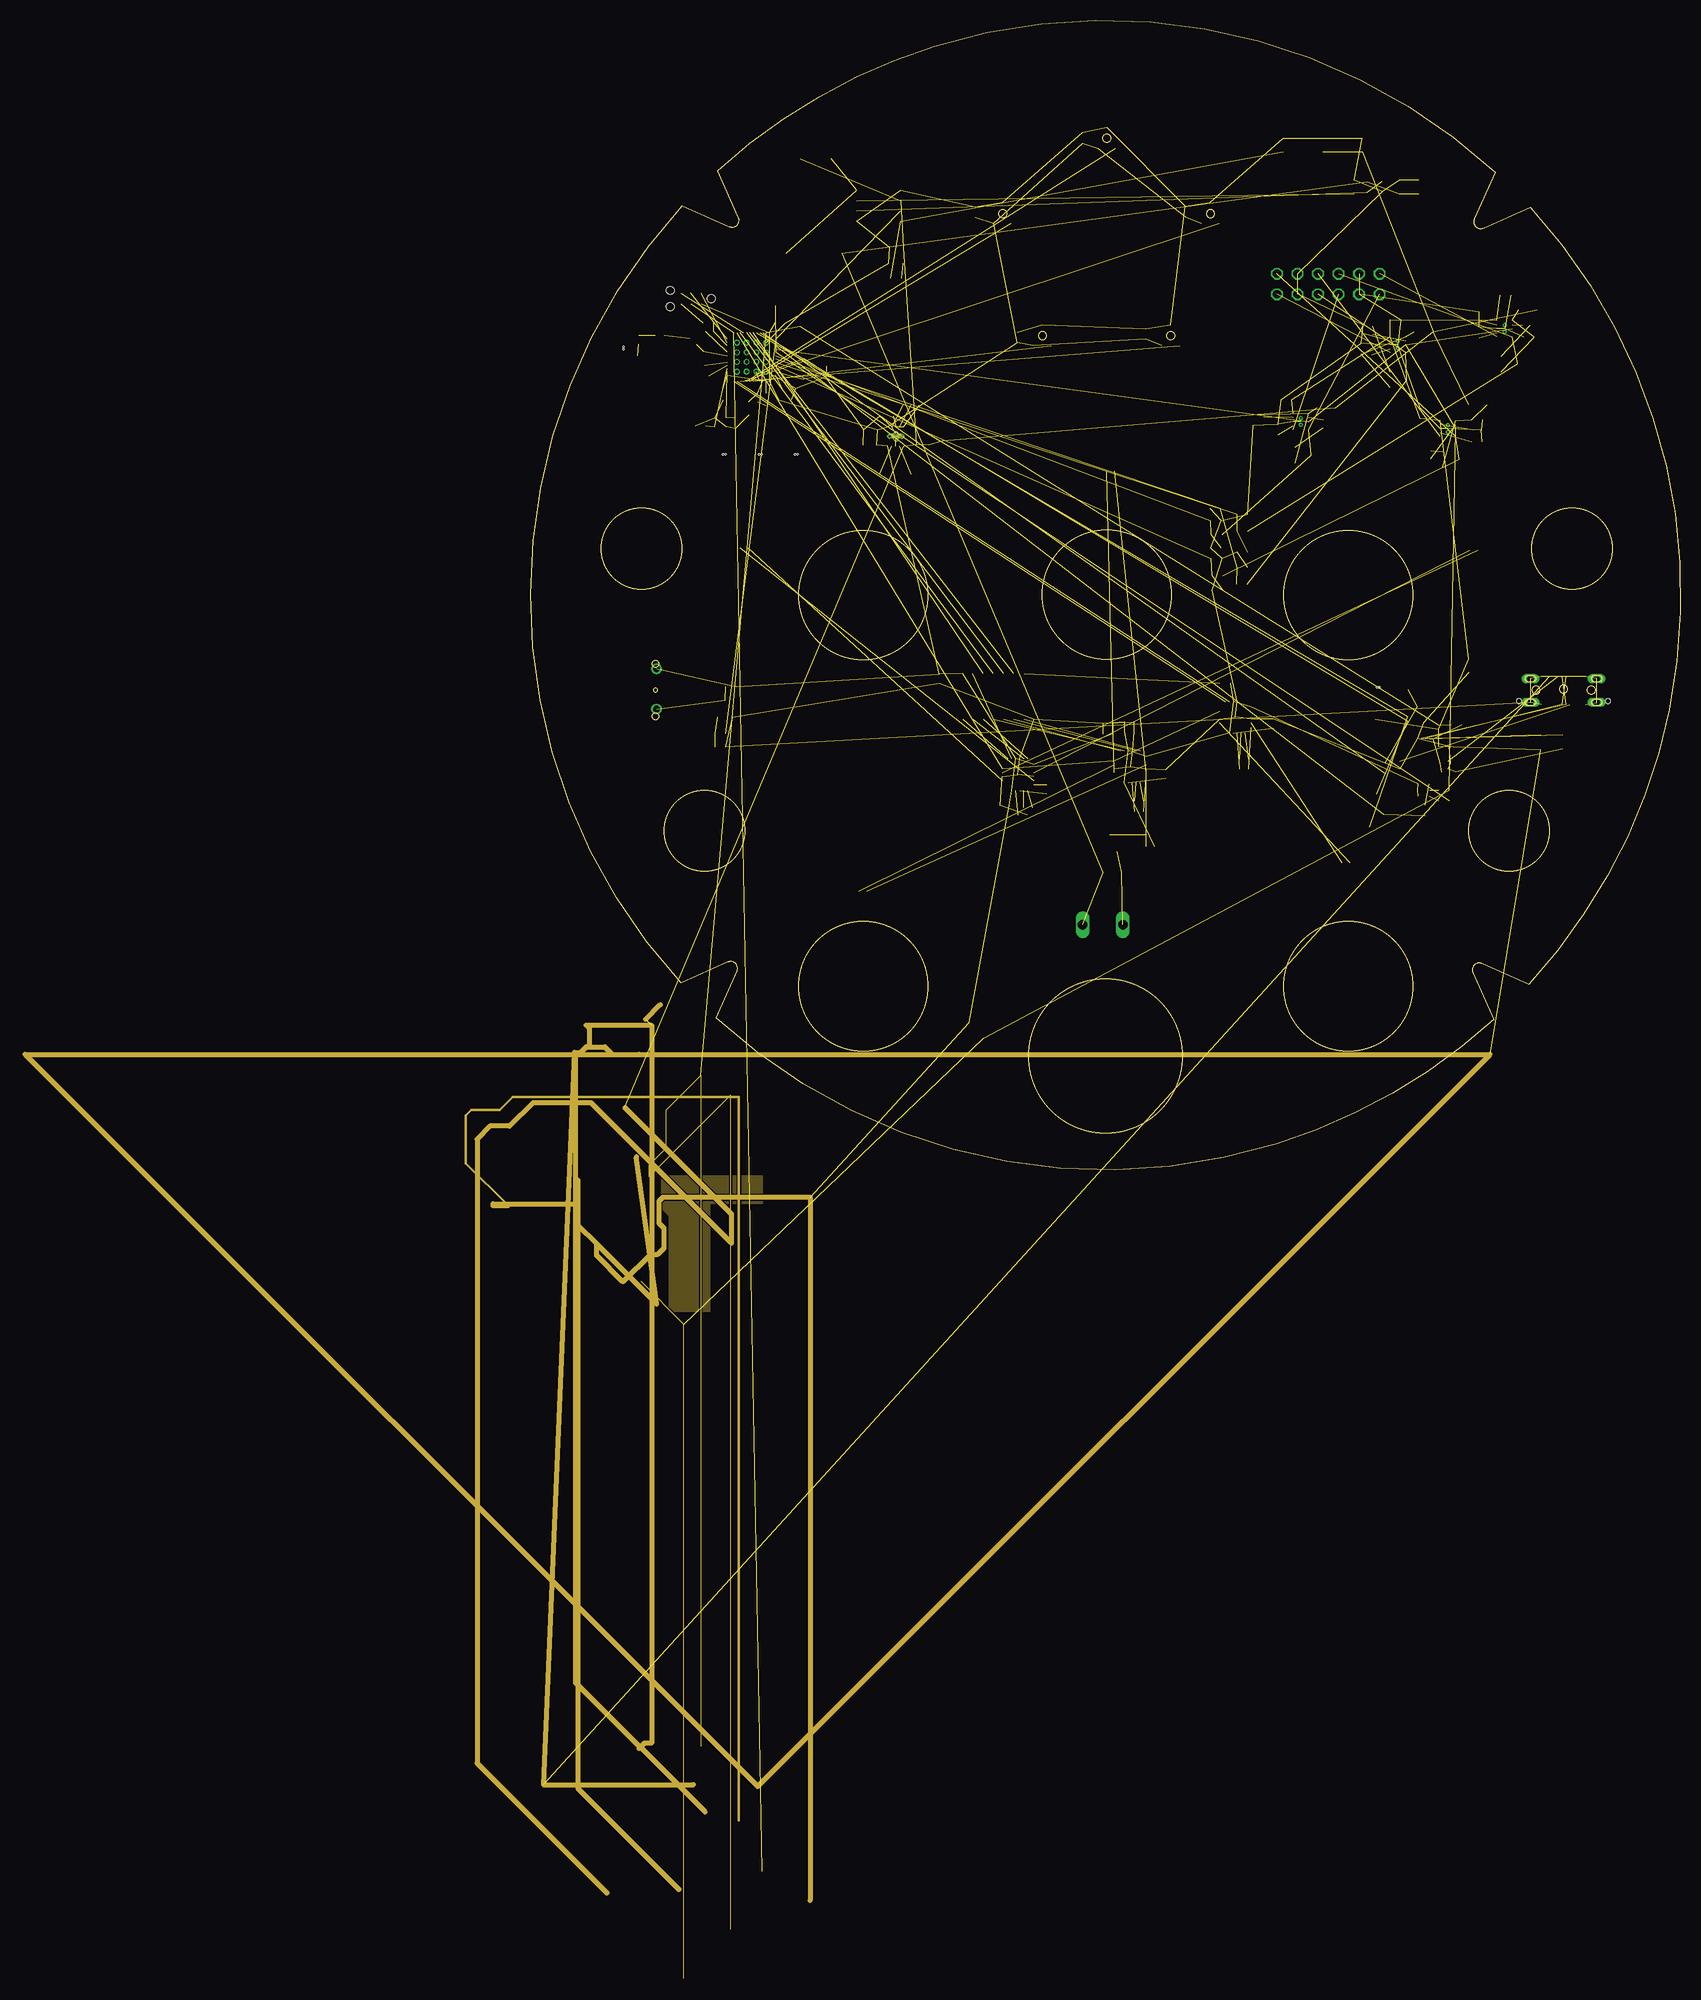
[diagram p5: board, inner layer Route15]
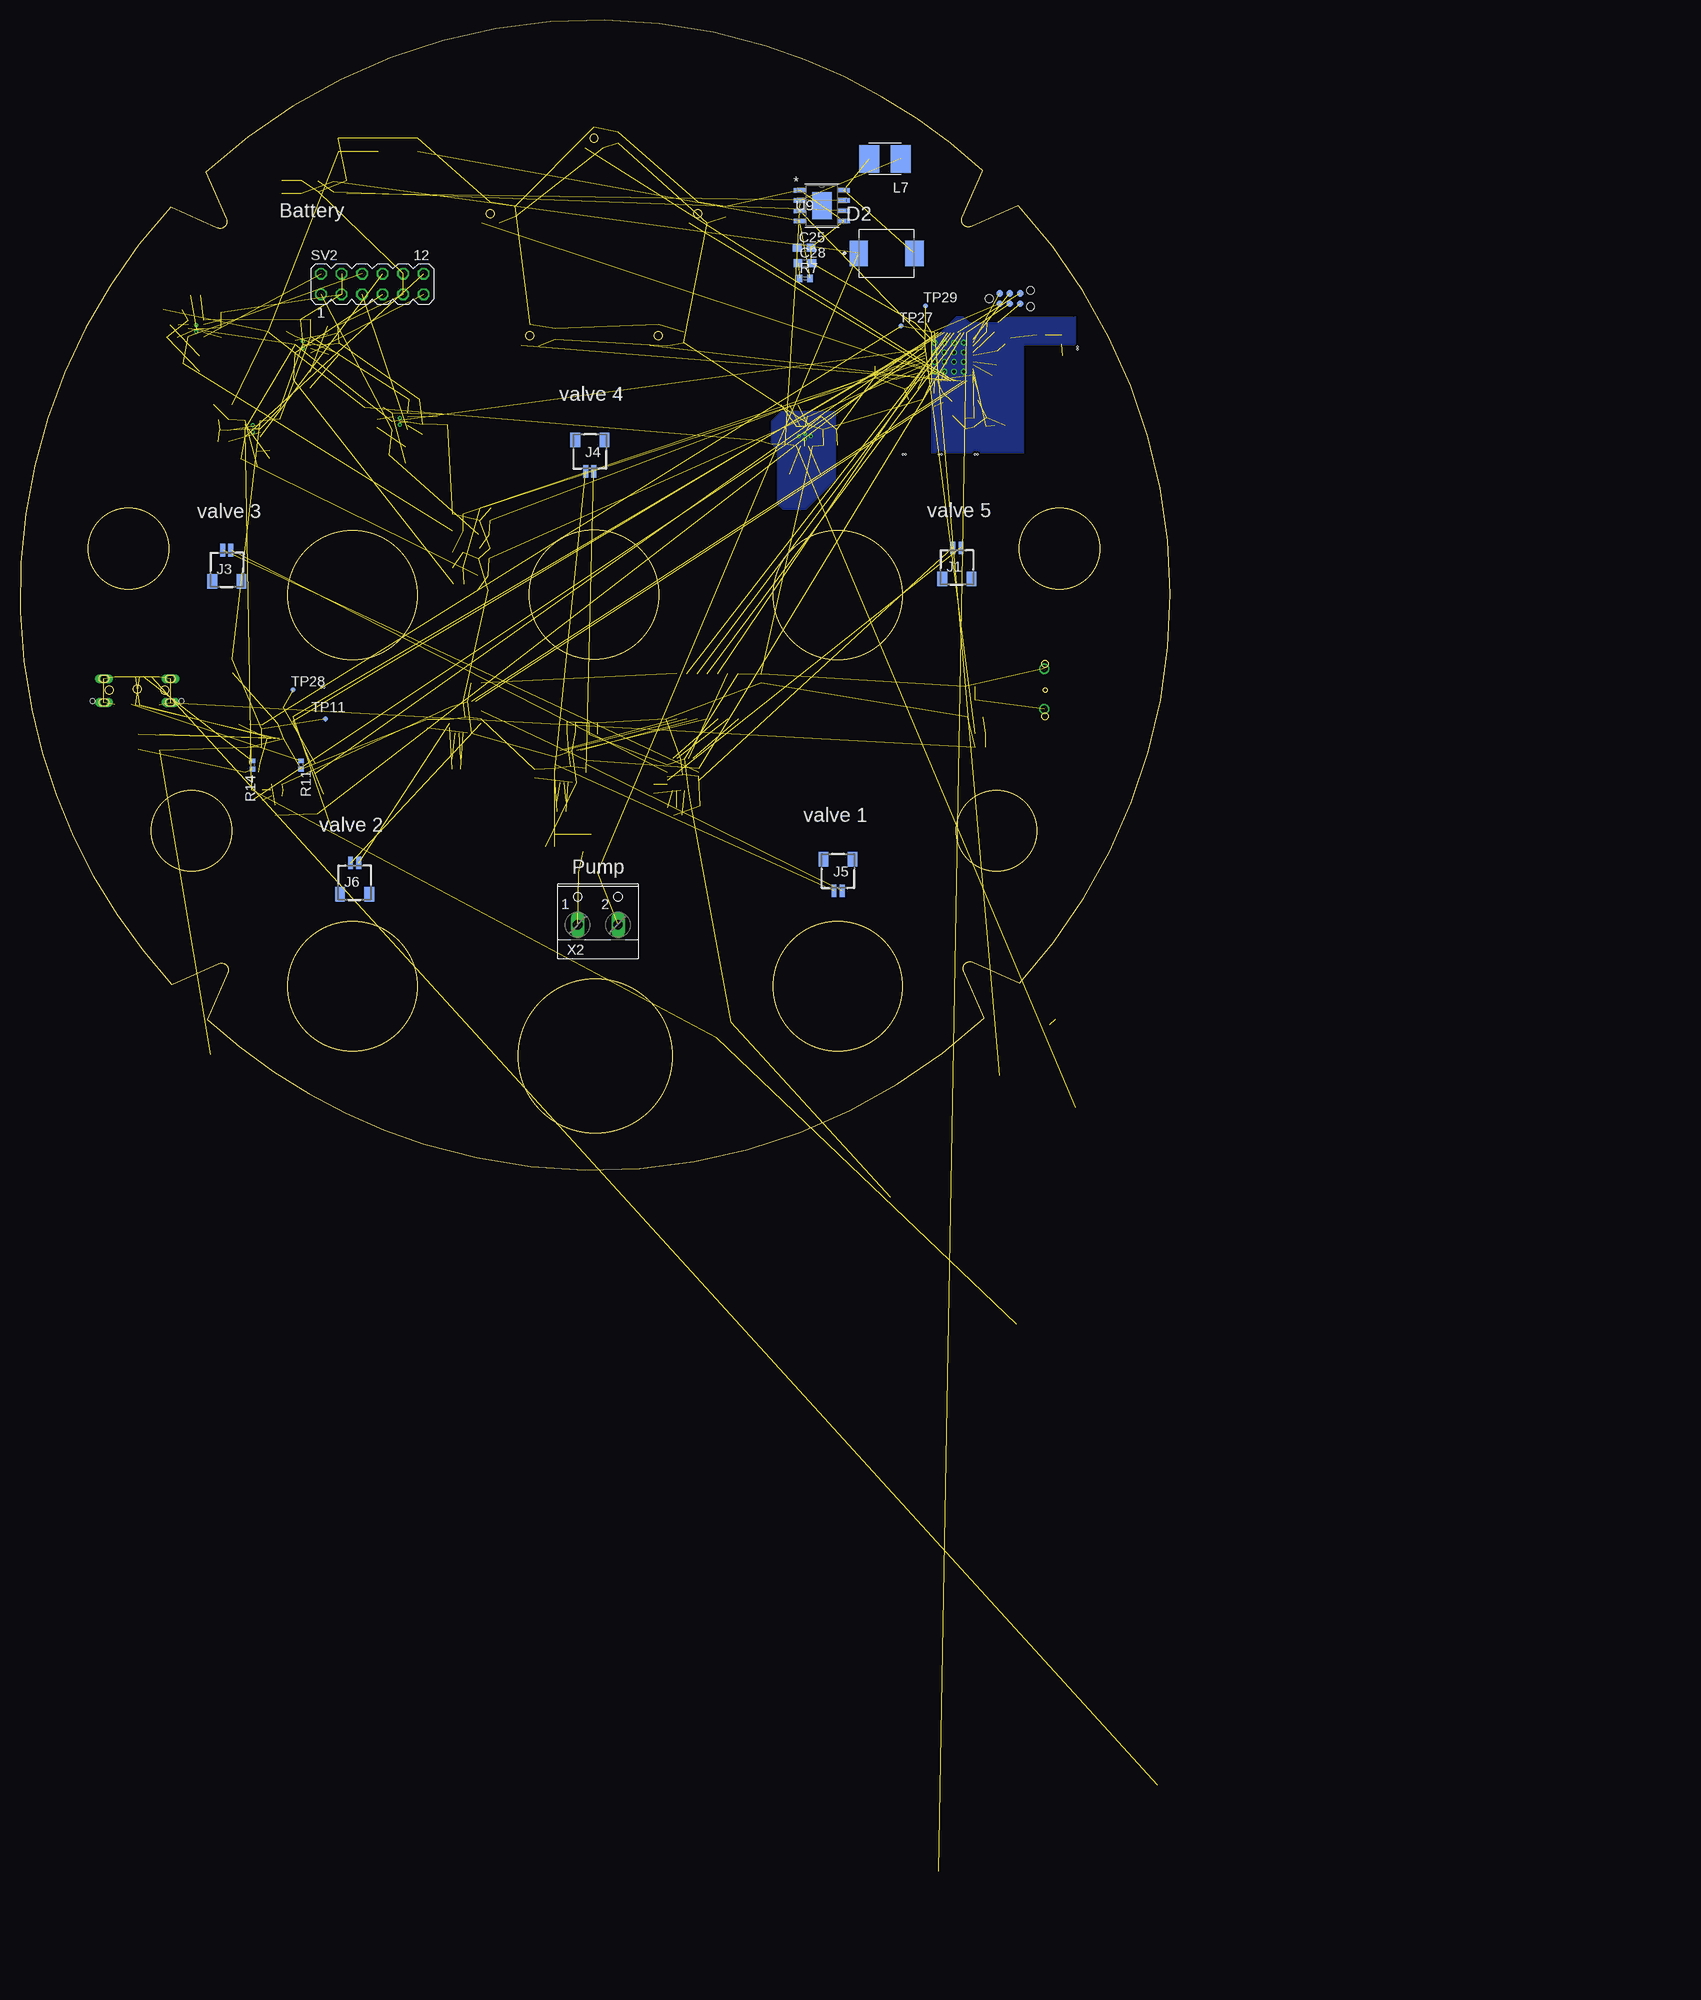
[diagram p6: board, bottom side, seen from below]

Size 142.25 x 142.25 mm. Coordinates in mm from the lower left corner, seen from the top.
Outline: 25.54,24.58 arc138 24.42,25.71
Outline: 18.62,23.14 arc-85 18.79,119.3
Outline: 24.6,116.72 arc138 25.73,117.85
Outline: 23.16,123.65 arc-25 49.95,139.03
Outline: 49.95,139.03 arc-60 119.31,123.46
Outline: 116.74,117.66 arc138 117.87,116.54
Outline: 123.66,119.1 arc-54 140.85,56.97
Outline: 140.85,56.97 arc-31 123.48,22.96
Outline: 117.68,25.53 arc138 116.56,24.4
Outline: 119.12,18.61 arc-25 92.32,3.22
Outline: 92.32,3.22 arc-60 22.97,18.77
Outline: 22.97,18.77 25.54,24.58
Outline: 25.54,24.58 arc138 24.42,25.71
Outline: 24.42,25.71 18.62,23.14
Outline: 18.62,23.14 arc-85 18.79,119.3
Outline: 18.79,119.3 24.6,116.72
Outline: 24.6,116.72 arc138 25.73,117.85
Outline: 25.73,117.85 23.16,123.65
Outline: 23.16,123.65 arc-25 49.95,139.03
Outline: 49.95,139.03 arc-60 119.31,123.46
Outline: 119.31,123.46 116.74,117.66
Outline: 116.74,117.66 arc138 117.87,116.54
Outline: 117.87,116.54 123.66,119.1
Outline: 123.66,119.1 arc-54 140.85,56.97
Outline: 140.85,56.97 arc-31 123.48,22.96
Outline: 123.48,22.96 117.68,25.53
Outline: 117.68,25.53 arc138 116.56,24.4
Outline: 116.56,24.4 119.12,18.61
Outline: 119.12,18.61 arc-25 92.32,3.22
Outline: 92.32,3.22 arc-60 22.97,18.77
Outline: circle at 79.2,103.23 radius 0.5
Outline: circle at 63.33,103.23 radius 0.5
Outline: circle at 58.43,118.32 radius 0.5
Outline: circle at 71.27,127.65 radius 0.5
Outline: circle at 84.11,118.32 radius 0.5
Outline: circle at 128.84,76.87 radius 5
Outline: circle at 121.05,41.96 radius 5
Outline: circle at 21.5,41.96 radius 5
Outline: circle at 13.71,76.87 radius 5
Outline: circle at 41.14,71.12 radius 8
Outline: circle at 71.28,71.17 radius 8
Outline: circle at 101.14,71.12 radius 8
Outline: circle at 101.14,22.72 radius 8
Outline: circle at 41.14,22.72 radius 8
Outline: circle at 71.12,14.1 radius 9.52
Outline: circle at 131.21,59.37 radius 0.5
Outline: circle at 124.37,59.37 radius 0.5
Outline: circle at 15.47,56.12 radius 0.4
Outline: circle at 15.47,62.62 radius 0.4
Outline: circle at 15.47,59.37 radius 0.25
Copper layers (1+2*15+16): Top 0.035mm / dielectric 0.213mm / Route2 0.035mm / dielectric 0.41mm / Route15 0.035mm / dielectric 0.213mm / Bottom 0.035mm
Design rules "default *": minimum track width 0.15mm, minimum drill 0.3mm, track to track 0.15mm, track to pad 0.15mm, pad to pad 0.15mm, via to via 0.15mm, smd to smd 0mil, copper to edge 0.3mm, drill to drill 0.3mm, minimum pad ring 0.15mm, minimum via ring 8mil, stop-mask expansion 0.025mm, vias tented up to drill 0.3mm, thermal gap 10mil
Holes 0.2 mm at 104.99,59.71 104.69,59.71 23.84,88.51 24.14,88.51 28.29,88.51 28.59,88.51 32.74,88.51 33.04,88.51 11.49,101.51 11.49,101.81

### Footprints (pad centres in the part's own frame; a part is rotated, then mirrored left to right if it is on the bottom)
C0402 = smd 0.7 x 0.9: 1 -0.65,0; 2 0.65,0
C0603 = smd 1.1 x 1: 1 -0.85,0; 2 0.85,0
RESC0402_N = smd 0.6 x 0.6: 1 -0.55,0; 2 0.55,0
LED_19-337C/RSBHGHC-A88/4T = smd 0.55 x 0.4: 1 0.675,0.725; 2 -0.675,0.725; 5 0.675,-0.725; 6 -0.675,-0.725 | smd 0.7 x 0.5: 3 0.75,0; 4 -0.75,0
DIOM7959X265N = smd 2.25 x 3.18: A 3.455,0; C -3.455,0
SOD-323 = smd 0.63 x 0.83: A 1.15,0; C -1.15,0
SOT23-W = smd 1.2 x 1.4: 1 -1.1,-1.3; 2 1.1,-1.3 | smd 1.8 x 1.2: 3 0,1.3
SM02B-SRSS-TB(LF)(SN) = smd 0.6 x 1.55: 1 -0.5,1.975; 2 0.5,1.975 | smd 1.2 x 1.8: 3 -1.8,-1.9; 4 1.8,-1.9
JAE_DX07S024WJ3R400 = smd 0.27 x 1.3: A1 -2.75,1.75; A2 -2.25,1.75; A3 -1.75,1.75; A4 -1.25,1.75; A5 -0.75,1.75; A6 -0.25,1.75; A7 0.25,1.75; A8 0.75,1.75; A9 1.25,1.75; A10 1.75,1.75; A11 2.25,1.75; A12 2.75,1.75; B1 2.75,-1.75; B2 2.25,-1.75; B3 1.75,-1.75; B4 1.25,-1.75; B5 0.75,-1.75; B6 0.25,-1.75; B7 -0.25,-1.75; B8 -0.75,-1.75; B9 -1.25,-1.75; B10 -1.75,-1.75; B11 -2.25,-1.75; B12 -2.75,-1.75 | drill 0.8 pad 1 long: S1 -4.1,1.47; S2 4.1,1.47; S3 4.1,-1.47; S4 -4.1,-1.47 | hole 0.6: -5.5,1.3; 5.5,1.3
SPARKFUN-JUMPERS_SMT-JUMPER_TRACE_SILK = smd 0.635 x 1.27: 1 -1.016,0; 2 0,0; 3 1.016,0
XFL4020 = smd 2.48 x 3.4: P$1 -1.93,0; P$2 1.93,0
RESC0603_N = smd 1.05 x 0.9: 1 -0.8,0; 2 0.8,0
XDCR_PS1240P02CT3 = drill 0.85 pad 1.28: 1 -2.5,0; 2 2.5,0
SOT23-3 = smd 0.8 x 0.9: 1 -0.95,-1; 2 0.95,-1; 3 0,1.1
R0402 = smd 0.7 x 0.9: 1 -0.65,0; 2 0.65,0
R0402' = smd 0.6 x 0.7: 1 -0.5,0; 2 0.5,0
MA06-2 = drill 1.016 octagon: 1 -6.35,-1.27; 2 -6.35,1.27; 3 -3.81,-1.27; 4 -3.81,1.27; 5 -1.27,-1.27; 6 -1.27,1.27; 7 1.27,-1.27; 8 1.27,1.27; 9 3.81,-1.27; 10 3.81,1.27; 11 6.35,-1.27; 12 6.35,1.27
SOT-23 = smd 0.787 x 0.889: 1 0.025,-1.016; 2 -0.94,1.016; 3 0.991,1.016
TP06R = smd 0.6 x 0.6: TP 0,0
SO16 = smd 0.6 x 1.2: 1 -4.445,-2.8; 2 -3.175,-2.8; 3 -1.905,-2.8; 4 -0.635,-2.8; 5 0.635,-2.8; 6 1.905,-2.8; 7 3.175,-2.8; 8 4.445,-2.8; 9 4.445,2.8; 10 3.175,2.8; 11 1.905,2.8; 12 0.635,2.8; 13 -0.635,2.8; 14 -1.905,2.8; 15 -3.175,2.8; 16 -4.445,2.8
QFN40P600X600X90-48_N = smd 0.65 x 0.2: 1 -3,2.2; 2 -3,1.8; 3 -3,1.4; 4 -3,1; 5 -3,0.6; 6 -3,0.2; 7 -3,-0.2; 8 -3,-0.6; 9 -3,-1; 10 -3,-1.4; 11 -3,-1.8; 12 -3,-2.2; 25 3,-2.2; 26 3,-1.8; 27 3,-1.4; 28 3,-1; 29 3,-0.6; 30 3,-0.2; 31 3,0.2; 32 3,0.6; 33 3,1; 34 3,1.4; 35 3,1.8; 36 3,2.2 | smd 0.2 x 0.65: 13 -2.2,-3; 14 -1.8,-3; 15 -1.4,-3; 16 -1,-3; 17 -0.6,-3; 18 -0.2,-3; 19 0.2,-3; 20 0.6,-3; 21 1,-3; 22 1.4,-3; 23 1.8,-3; 24 2.2,-3; 37 2.2,3; 38 1.8,3; 39 1.4,3; 40 1,3; 41 0.6,3; 42 0.2,3; 43 -0.2,3; 44 -0.6,3; 45 -1,3; 46 -1.4,3; 47 -1.8,3; 48 -2.2,3 | smd 4.7 x 4.7: PAD 0,0 | drill 0.4: PAD@VIA01 -1.8,1.8; PAD@VIA02 -1.8,0.6; PAD@VIA03 -1.8,-0.6; PAD@VIA04 -1.8,-1.8; PAD@VIA05 -0.6,1.8; PAD@VIA06 -0.6,0.6; PAD@VIA07 -0.6,-0.6; PAD@VIA08 -0.6,-1.8; PAD@VIA09 0.6,1.8; PAD@VIA10 0.6,0.6; PAD@VIA11 0.6,-0.6; PAD@VIA12 0.6,-1.8; PAD@VIA13 1.8,1.8; PAD@VIA14 1.8,0.6; PAD@VIA15 1.8,-0.6; PAD@VIA16 1.8,-1.8
QFN50P400X400X100-25N = smd 0.81 x 0.26: 1 -1.955,1.25; 2 -1.955,0.75; 3 -1.955,0.25; 4 -1.955,-0.25; 5 -1.955,-0.75; 6 -1.955,-1.25; 13 1.955,-1.25; 14 1.955,-0.75; 15 1.955,-0.25; 16 1.955,0.25; 17 1.955,0.75; 18 1.955,1.25 | smd 0.26 x 0.81: 7 -1.25,-1.955; 8 -0.75,-1.955; 9 -0.25,-1.955; 10 0.25,-1.955; 11 0.75,-1.955; 12 1.25,-1.955; 19 1.25,1.955; 20 0.75,1.955; 21 0.25,1.955; 22 -0.25,1.955; 23 -0.75,1.955; 24 -1.25,1.955 | smd 2.8 x 2.8: 25 0,0
QFN50P400X400X80-25N = smd 0.84 x 0.26: 1 -1.935,1.25; 2 -1.935,0.75; 3 -1.935,0.25; 4 -1.935,-0.25; 5 -1.935,-0.75; 6 -1.935,-1.25; 13 1.935,-1.25; 14 1.935,-0.75; 15 1.935,-0.25; 16 1.935,0.25; 17 1.935,0.75; 18 1.935,1.25 | smd 0.26 x 0.84: 7 -1.25,-1.935; 8 -0.75,-1.935; 9 -0.25,-1.935; 10 0.25,-1.935; 11 0.75,-1.935; 12 1.25,-1.935; 19 1.25,1.935; 20 0.75,1.935; 21 0.25,1.935; 22 -0.25,1.935; 23 -0.75,1.935; 24 -1.25,1.935 | smd 2.45 x 2.45: 25 0,0
SOT143 = smd 1.4 x 1.1: 1 -1.35,0.86 | smd 1.4 x 0.9: 2 -1.35,-0.96; 3 1.35,-0.96; 4 1.35,0.96
SON50P250X250X80-11N = smd 0.84 x 0.27: 1 -1.195,1; 2 -1.195,0.5; 3 -1.195,0; 4 -1.195,-0.5; 5 -1.195,-1; 6 1.195,-1; 7 1.195,-0.5; 8 1.195,0; 9 1.195,0.5; 10 1.195,1 | smd 1.2 x 2: 11 0,0 | drill 0.2 pad 0.3: 12 0.35,0; 13 -0.35,0; 14 0,0.75; 15 0,-0.75
SOP-8_PAM2423AECADJR_DIO = smd 1.462 x 0.559: 1 -2.725,1.905; 2 -2.725,0.635; 3 -2.725,-0.635; 4 -2.725,-1.905; 5 2.725,-1.905; 6 2.725,-0.635; 7 2.725,0.635; 8 2.725,1.905 | smd 2.413 x 3.302: EPAD 0,0
TEXAS_INSTRUMENTS_BQ25050DQCR_0 = smd 0.5 x 0.25: 1 -0.95,1; 2 -0.95,0.5; 3 -0.95,0; 4 -0.95,-0.5; 5 -0.95,-1; 6 0.95,-1; 7 0.95,-0.5; 8 0.95,0; 9 0.95,0.5; 10 0.95,1 | smd 0.84 x 2.4: 11 0,0 | drill 0.2 pad 0.5: PAD_1 0,0.416; PAD_2 0,-0.416
J-LINK_6-PIN_ADAPTER_S = smd 0.787 x 0.787: P$1 -1.27,-0.635; P$2 -1.27,0.635; P$3 0,-0.635; P$4 0,0.635; P$5 1.27,-0.635; P$6 1.27,0.635 | hole 0.991: -2.54,0; 2.54,1.016; 2.54,-1.016
2450AT18B100E = smd 1 x 1.6: P$1 -1.6,0; P$2 1.6,0
W237-102 = drill 1.194 long: 1 -2.5,-1.27; 2 2.5,-1.27
BT-XTAL_2016_N = smd 0.95 x 0.85: 1 -0.725,-0.575; 2 0.725,-0.575; 3 0.725,0.575; 4 -0.725,0.575
XTAL_3215_N = smd 1 x 1.8: 1 -1.25,0; 2 1.25,0

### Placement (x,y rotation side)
C1  60.19,103.01 90 top
C2  41.99,89.66 180 top
C3  54.99,118.51 90 top
C4  68.29,127.71 90 top
C5  113.19,50.36 180 top
C6  113.59,49.21 0 top
C7  42.09,91.61 180 top
C8  80.99,118.61 90 top
C9  44.04,93.26 0 top
C10  76.09,103.41 90 top
C11  50.59,60.81 90 top
C12  116.04,62.36 90 top
C13  25.3,92.35 270 top
C14  21.04,92.11 180 top
C15  21.86,101.79 45 top
C16  31.99,96.66 0 top
C17  30.89,104.76 0 top
C18  20.69,99.56 180 top
C19  21.39,98.26 180 top
C20  23.79,95.91 270 top
C21  31.49,95.31 0 top
C22  26.99,94.21 270 top
C23  35.89,98.11 180 top
C24  35.91,99.42 180 top
C25  45.29,114.11 0 bottom
C26  47.69,90.66 90 top
C27  113,52.4 0 top
C28  45.19,112.21 0 bottom
C29  93.09,126.81 90 top
C30  97.99,126.81 90 top
C31  61.59,44.81 180 top
C32  63.89,47.11 90 top
C33  60.89,43.91 180 top
C34  110.09,93.61 90 top
C35  15.99,103.26 0 top
C36  49.24,90.61 90 top
C37  50.94,91.06 90 top
C38  21.99,104.81 180 top
C39  117.09,92.81 180 top
C40  58.69,45.11 180 top
C41  117.09,90.11 180 top
C42  120.59,108.21 0 top
C43  123.49,103.01 0 top
C44  117.39,103.61 270 top
C45  106.99,105.21 0 top
C46  102.79,101.61 270 top
C47  104.09,101.51 270 top
C48  93.49,95.31 180 top
C49  89.39,92.81 90 top
C50  92.49,91.61 270 top
C51  102.89,126.81 90 top
C52  101.89,121.61 90 top
C53  109.89,121.61 90 top
C54  76.69,40.01 0 top
C55  88.29,50.81 180 top
C56  88.29,49.61 0 top
C57  91.89,55.21 270 top
C58  74.09,54.21 0 top
C59  74.09,55.41 180 top
C60  75.29,45.61 180 top
C61  75.29,44.31 0 top
C62  78.59,49.01 270 top
C63  71.39,53.91 180 top
C64  71.39,55.31 0 top
C65  107.49,121.61 90 top
C66  88.09,81.11 0 top
C67  88.09,74.51 0 top
C68  84.79,80.31 0 top
C69  84.89,75.61 0 top
D1  110.49,47.01 0 top
D2  35.09,113.41 0 bottom
D3  71.99,36.81 0 top
D4  123.39,106.41 180 top
D5  117.19,94.71 0 top
D6  110.49,103.71 180 top
D7  98.49,94.31 180 top
IC1  63.29,103.31 0 top
IC2  58.39,118.41 0 top
IC3  71.29,127.71 0 top
IC4  84.09,118.41 0 top
IC5  79.19,103.31 0 top
J1  26.39,75.01 0 bottom
J2  127.79,59.31 180 top
J3  116.69,74.71 0 bottom
J4  71.79,88.41 180 bottom
J5  41.09,36.51 180 bottom
J6  100.89,36.01 0 bottom
JP1  47.09,94.61 0 top
L1  45.14,86.11 0 top
L2  20.09,102.53 135 top
L3  29.19,95.31 270 top
L4  28.09,95.56 90 top
L5  14.49,103.81 270 top
L6  13.39,102.71 90 top
L7  35.29,125.11 180 bottom
LS1  15.59,59.51 90 top
Q1  24.09,57.01 0 top
Q2  72.59,40.51 180 top
R1  85.89,60.21 0 top
R2  110.69,44.51 270 top
R3  75.49,41.51 0 top
R4  112.99,47.01 0 top
R5  1k  [R0402']  117.09,91.51 180 top
R6  24.79,59.81 180 top
R7  45.19,110.31 0 bottom
R8  105.74,49.66 270 top
R9  103.49,121.61 90 top
R10  112.99,45.71 0 top
R11  5.1k  [R0402']  107.54,50.11 90 bottom
R12  105.39,121.71 90 top
R13  23.49,54.01 180 top
R14  5.1k  [R0402']  113.54,50.11 270 bottom
R15  23.49,52.31 0 top
R16  114.54,55.11 180 top
R17  1k  [R0402']  111.39,88.51 270 top
R18  1k  [R0402']  117.39,105.61 270 top
R19  1k  [R0402']  22.19,103.71 180 top
R20  1k  [R0402']  123.19,104.51 180 top
R21  1k  [R0402']  102.99,104.01 270 top
R22  1k  [R0402']  104.19,103.91 270 top
R23  1k  [R0402']  90.69,92.71 90 top
R24  1k  [R0402']  98.09,92.31 90 top
R25  88.09,79.01 0 top
R26  88.09,76.41 0 top
R27  87.99,72.51 0 top
R28  84.69,81.91 0 top
R29  84.89,78.61 0 top
R30  84.79,76.91 0 top
R31  84.99,73.51 0 top
R32  84.99,71.71 0 top
SV2  98.69,109.61 0 bottom
T1  113.89,87.91 90 top
T2  121.09,99.71 90 top
T3  107.39,97.71 90 top
T4  95.59,88.41 90 top
TP11  104.49,55.81 0 bottom
TP14  54.29,18.21 0 top
TP21  104.69,46.51 0 top
TP22  103.79,42.41 0 top
TP27  33.29,104.41 0 bottom
TP28  108.49,59.41 0 bottom
TP29  30.29,106.91 0 bottom
TP30  56.09,16.31 0 top
TP31  105.49,44.01 0 top
U1  57.89,58.61 0 top
U2  27.34,100.56 180 top
U3  60.29,48.91 0 top
U4  87.19,56.01 0 top
U5  110.44,55.31 90 top
U6  126.32,52.91 180 top
U7  74.19,49.91 0 top
U8  45.19,90.76 90 top
U9  43.09,119.31 0 bottom
U10  120.49,104.11 0 top
U11  113.49,91.71 0 top
U12  107.29,102.11 0 top
U13  95.29,92.61 0 top
U$1  19.82,107.81 0 bottom
U$16  13.29,99.16 270 top
X2  70.79,31.61 0 bottom
X3  23.49,92.51 0 top
X4  33.81,99.11 90 top

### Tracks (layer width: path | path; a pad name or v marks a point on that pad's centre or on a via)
3.3V  (45 unrouted)
  Route15 0.305: -2.78,-4.42 -8.01,0.81 -8.01,6.71 -7.31,7.41 -3.81,7.41 -2.21,9.01 25.74,9.01 25.74,-80.49
  Route15 0.61: -2.78,-4.42 -4.65,-4.4 -4.65,-4.2 5.87,-4.2 | 8.19,-9.19 8.19,-10.59 11.44,-13.84 14.85,-10.43 15.75,-10.43 16.49,-9.69 16.49,-7.19 15.89,-6.59 15.89,-3.89 16.39,-3.39 34.59,-3.39 34.59,-90.39 | 5.87,-4.2 5.87,-6.88 8.19,-9.19 | 5.87,-4.2 5.87,-2.58 | 18.39,-89.04 5.87,-76.53 5.87,-4.38 5.87,-2.58 | 13.09,1.61 15.6,-16.6 8.19,-9.19 | 5.87,-1.3 5.87,-2.58
12V  (5 unrouted)
ANT1  (2 unrouted)
BAT0  (3 unrouted)
BAT1  (3 unrouted)
BAT2  (3 unrouted)
BAT3  (3 unrouted)
BAT_ADC_0  (3 unrouted)
BAT_ADC_1  (3 unrouted)
BAT_ADC_2  (3 unrouted)
BAT_ADC_3  (3 unrouted)
BT_HALL  (1 unrouted)
BUZZER  (1 unrouted)
CLOCK  (1 unrouted)
DATA  (1 unrouted)
DEC1  (1 unrouted)
DEC2  (1 unrouted)
DEC3  (1 unrouted)
DEC4  (2 unrouted)
DN  (3 unrouted)
DP  (3 unrouted)
EN_OUT  (1 unrouted)
GND  (121 unrouted)
  Route15 0.61: U8.15 U8.14 | U8.13 U8.12
  cutout Route15: 4.44,21.41 4.44,19.11 3.09,19.11 3.09,21.41
  cutout Route15: 13.09,17.26 13.09,14.91 11.74,14.91 11.74,17.26
  cutout Route15: 13.04,21.41 13.04,19.11 11.79,19.11 11.79,21.41
  cutout Route15: 4.44,17.26 4.44,14.86 3.09,14.86 3.09,17.26
  pour Route2 (no thermals): -2.96,22.41 -8.81,16.56 -8.81,7.96 -9.16,7.61 -10.61,7.61 -11.21,7.01 -11.21,-1.24 -11.71,-1.74 -14.31,-1.74 -15.01,-2.44 -15.01,-8.89 -6.76,-17.14 22.19,-17.14 22.19,-4.39 22.29,-4.29 28.69,-4.29 28.69,-1.29 24.79,-1.29 24.79,7.91 22.69,7.91 22.69,16.71 16.99,22.41
  pour Bottom (no thermals): 41.39,85.46 41.39,93.81 48.14,93.81 49.34,92.61 49.34,90.01 48.59,89.26 48.59,82.51 47.84,81.76 45.09,81.76
  pour Top (no thermals): 46.09,90.16 46.89,90.96 49.54,90.96 50.04,91.46 51.09,91.46 51.14,91.51 51.14,92.56 50.09,92.56 49.59,92.06 47.06,92.06 46.31,91.31 43.94,91.31 43.84,91.21 43.84,90.41 44.04,90.21 46.04,90.21
  pour Top (isolate 0.2, no thermals): 25.19,88.71 25.19,91.41 24.99,91.61 19.99,91.61 19.69,91.91 19.69,94.51 20.59,94.51 20.59,99.81 25.19,99.81 25.19,104.66 24.19,105.66 11.69,105.66 11.69,102.06 18.19,102.06 18.19,88.71
  pour Bottom: 29.44,88.66 29.44,102.51 26.39,105.56 25.64,105.56 24.89,104.81 21.19,104.81 20.49,105.51 11.74,105.56 11.74,102.06 18.19,102.06 18.19,88.66
  pour Route15: 22.19,-17.59 17.19,-17.59 17.14,-12.54 17.14,-5.69 16.24,-4.79 16.24,-1.14 16.69,-0.69 28.69,-0.69 28.69,-4.24 22.19,-4.24
  cutout Top: 16.59,103.66 16.59,102.86 15.39,102.86 15.39,103.66
  cutout Top: 14.59,103.66 14.59,102.86 13.39,102.86 13.39,103.66
  cutout Top: 13.78,102.13 12.98,102.13 12.98,103.33 13.78,103.33
  cutout Top: 21.79,92.36 21.79,91.46 20.39,91.46 20.39,92.36
  cutout Top: 19.89,103.31 21.59,101.61 21.04,101.06 19.34,102.76
I_HALL  (1 unrouted)
II_HALL  (1 unrouted)
III_HALL  (1 unrouted)
IN1A  (1 unrouted)
IN1B  (1 unrouted)
IN2A  (1 unrouted)
IN2B  (1 unrouted)
IN3A  (1 unrouted)
IN3B  (1 unrouted)
IN4A  (1 unrouted)
IN4B  (1 unrouted)
IN5A  (1 unrouted)
IN5B  (1 unrouted)
ISENSE0  (1 unrouted)
ISENSE1  (1 unrouted)
ISENSE2  (1 unrouted)
ISENSE3  (1 unrouted)
LED_B  (2 unrouted)
LED_G  (2 unrouted)
LED_R  (7 unrouted)
  Route15 0.152: 13.69,-13.79 18.99,-19.09 18.99,-99.99
N$1  (2 unrouted)
N$2  (1 unrouted)
N$3  (2 unrouted)
N$4  (1 unrouted)
N$5  (1 unrouted)
N$6  (3 unrouted)
N$7  (1 unrouted)
  pour Top (no thermals): 48.14,84.46 45.99,84.46 45.54,84.91 45.54,88.91 45.59,88.96 45.84,88.96 47.04,87.76 47.89,87.76 48.14,87.51
N$8  (1 unrouted)
N$9  (1 unrouted)
N$10  (1 unrouted)
N$11  (1 unrouted)
  pour Top (no thermals): 44.99,88.71 44.99,84.81 44.64,84.46 43.54,84.46 43.24,84.76 43.24,87.46 44.49,88.71
N$12  (2 unrouted)
N$13  (1 unrouted)
N$14  (2 unrouted)
N$15  (1 unrouted)
N$16  (2 unrouted)
N$17  (1 unrouted)
N$18  (2 unrouted)
N$19  (1 unrouted)
N$20  (1 unrouted)
N$21  (1 unrouted)
N$23  (1 unrouted)
N$24  (1 unrouted)
N$26  (3 unrouted)
N$27  (1 unrouted)
N$28  (1 unrouted)
N$29  (2 unrouted)
N$30  (1 unrouted)
N$31  (3 unrouted)
N$33  (1 unrouted)
N$34  (1 unrouted)
N$36  (1 unrouted)
N$37  (3 unrouted)
N$39  (2 unrouted)
N$40  (1 unrouted)
N$41  (1 unrouted)
N$43  (1 unrouted)
N$44  (1 unrouted)
N$45  (1 unrouted)
N$46  (1 unrouted)
N$47  (1 unrouted)
N$48  (2 unrouted)
N$50  (1 unrouted)
N$51  (1 unrouted)
N$52  (1 unrouted)
N$53  (1 unrouted)
N$54  (1 unrouted)
N$55  (1 unrouted)
N$56  (3 unrouted)
N$58  (1 unrouted)
N$59  (1 unrouted)
N$60  (1 unrouted)
N$61  (1 unrouted)
N$62  (1 unrouted)
N$63  (1 unrouted)
N$64  (1 unrouted)
ON_HALL  (1 unrouted)
OUT1A  (1 unrouted)
OUT1B  (1 unrouted)
OUT2A  (1 unrouted)
OUT2B  (1 unrouted)
OUT3A  (1 unrouted)
OUT3B  (1 unrouted)
OUT4A  (1 unrouted)
OUT4B  (1 unrouted)
OUT5A  (1 unrouted)
OUT5B  (1 unrouted)
P0.00/XL1  (2 unrouted)
P0.01/XL2  (2 unrouted)
P0.22  (2 unrouted)
P0.24  (1 unrouted)
PSAVE  (3 unrouted)
PUMP  (1 unrouted)
PWR_EN_1  (1 unrouted)
RCK  (1 unrouted)
RST_CP  (4 unrouted)
  Route15 0.15: 24.76,-93.94 24.76,9.28 14.69,-0.79 14.69,0.63 16.79,2.73 16.79,7.39 21.09,11.69 21.09,-71.29
RST_NRF  (2 unrouted)
  Route2 0.305: 32.44,-90.59 28.64,-86.79 27.84,-86.79
RXD  (2 unrouted)
SUSPEND  (1 unrouted)
SWCLK  (1 unrouted)
SWDIO  (1 unrouted)
SWO  (1 unrouted)
TS0  (1 unrouted)
TS1  (1 unrouted)
TS2  (1 unrouted)
TS3  (1 unrouted)
TXD  (2 unrouted)
VBUS  (16 unrouted)
  Route15 0.61: 5.41,14.53 5.41,14.55 5.55,14.41 5.55,-63.41 21.59,-79.44 | 20.17,-76.07 1.6,-76.07 5.41,14.53 | 13.44,14.31 -62.51,14.31 28.09,-76.29 118.69,14.31 10.09,14.31 9.19,15.21 7.29,15.21 | 14.23,18.63 16.07,20.46 | 5.41,14.53 6.21,14.53 6.89,15.21 7.29,15.21 | 7.29,15.21 7.29,17.51 6.89,17.91 14.99,17.91 14.99,-70.94 14.09,-70.94 13.44,-71.59
VCC  (13 unrouted)
  Route15 0.61: 9.49,-89.49 -6.61,-73.39 -6.61,3.81 -5.01,5.41 -2.57,5.41 0.33,8.31 7.49,8.31 24.84,-9.04 24.84,-5.44 11.69,7.71
VDD  (4 unrouted)
X2  (2 unrouted)

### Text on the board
bNames: Battery | valve 4 | valve 5 | valve 3 | valve 1 | valve 2 | Pump

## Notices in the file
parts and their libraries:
SparkFun-PowerSymbols: Licensing: Creative Commons ShareAlike 4.0 International - https://creativecommons.org/licenses/by-sa/4.0
